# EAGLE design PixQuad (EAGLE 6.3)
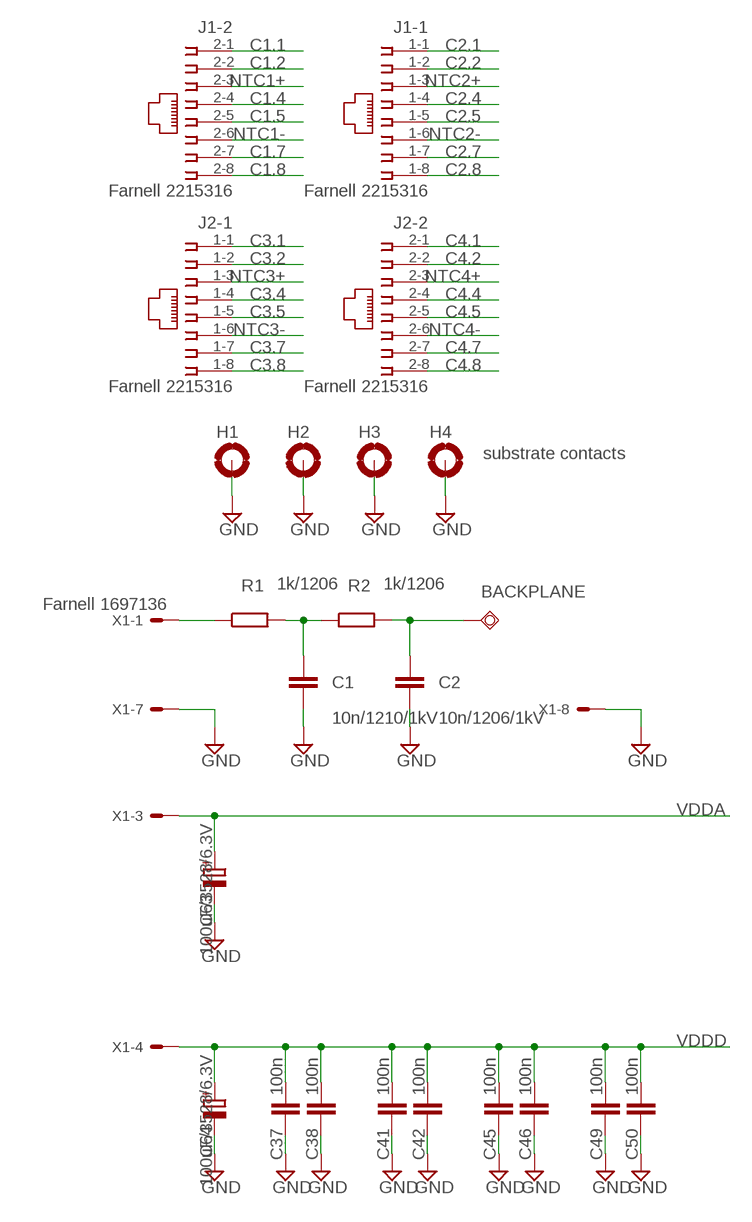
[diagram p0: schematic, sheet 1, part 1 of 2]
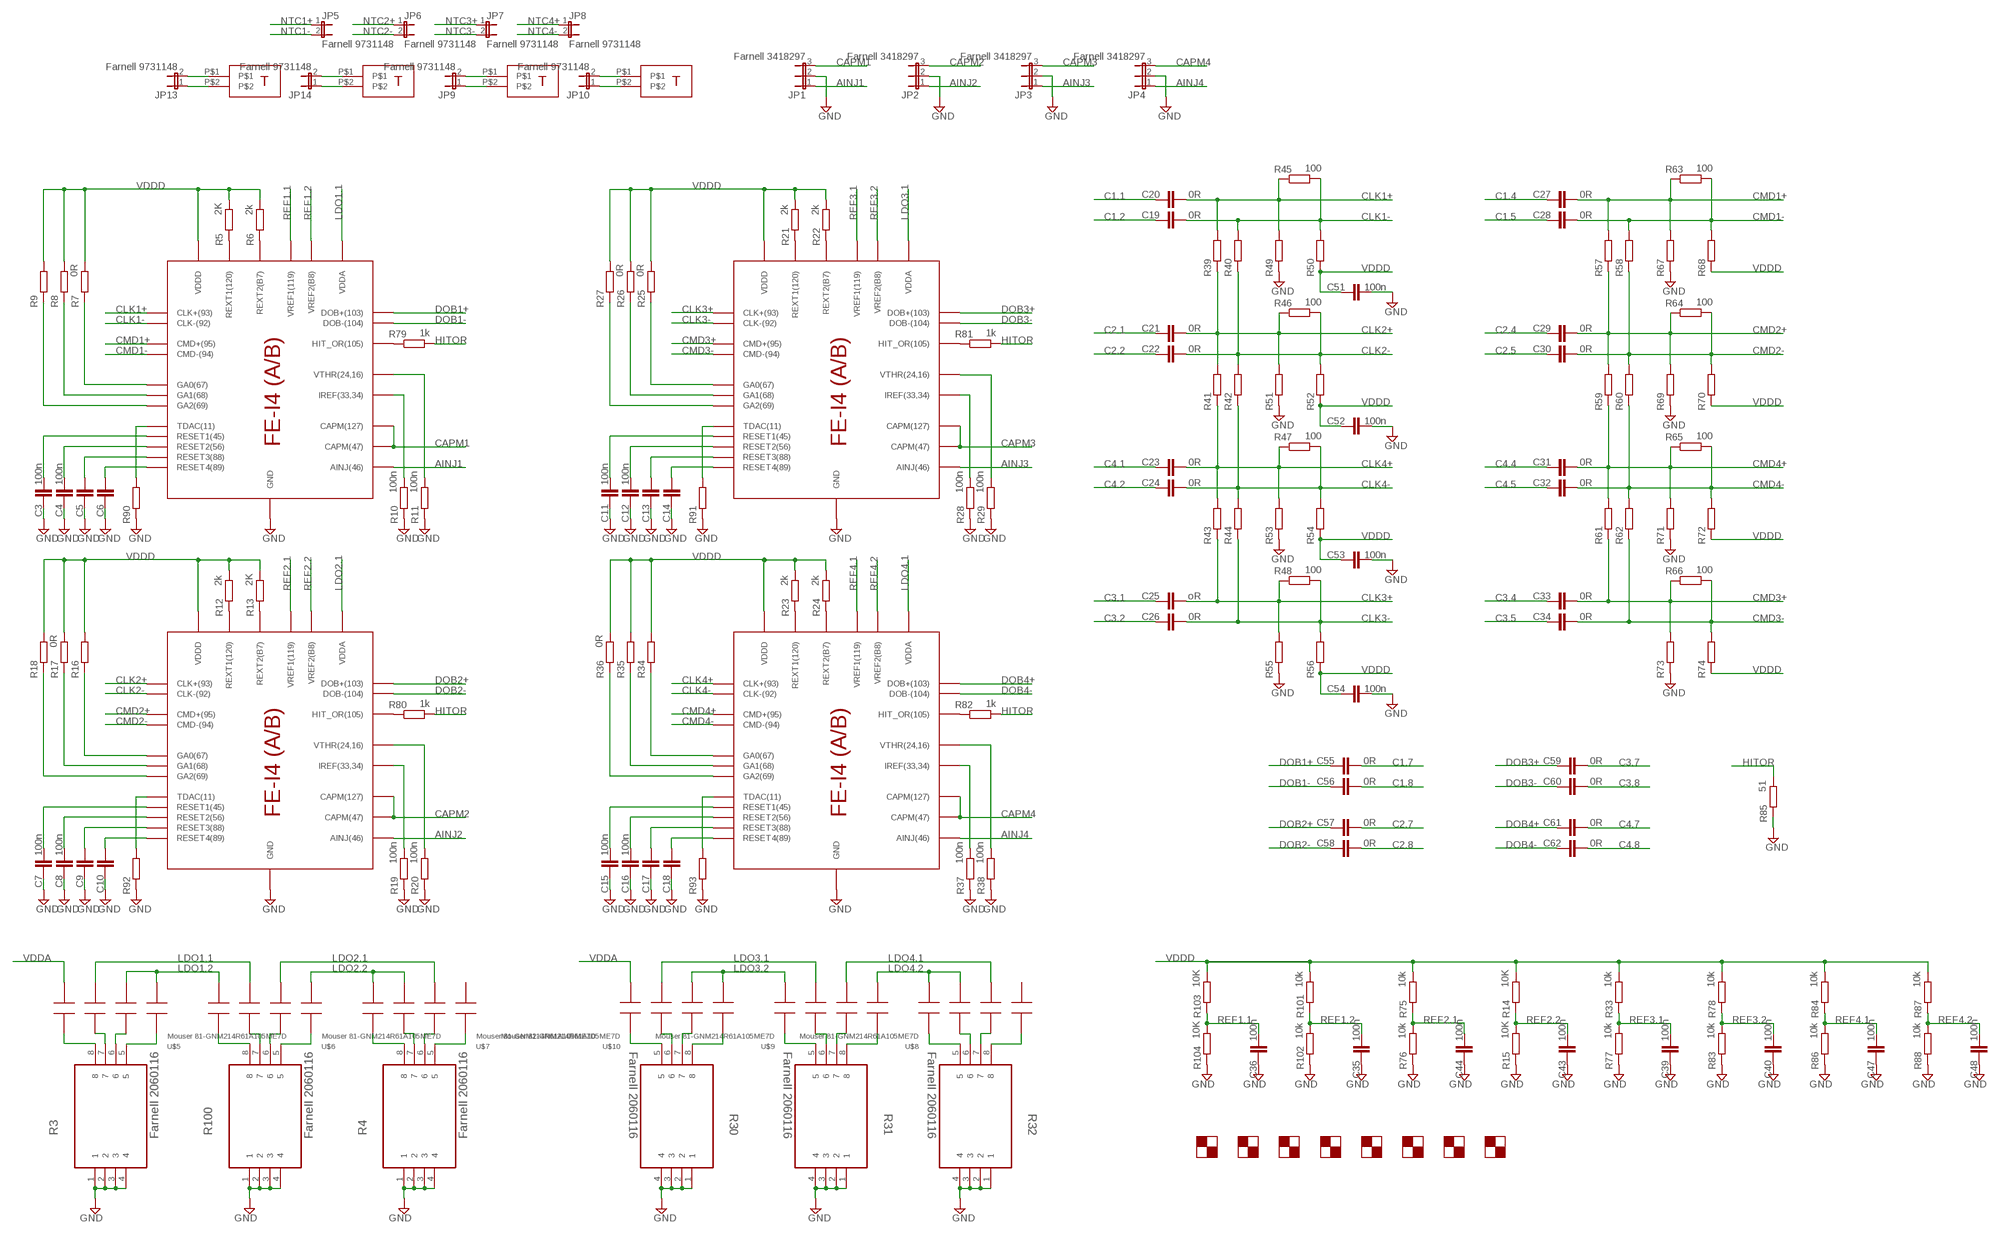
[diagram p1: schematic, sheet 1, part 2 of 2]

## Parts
BACKPLANE  TPSQTP20SQ  [TP20SQ]
C1  10n/1210/1kV  C-EUC1210  [C1210]
C2  10n/1206/1kV  C-EUC1210  [C1210]
C3  100n  C-EUC0402  [C0402]
C4  100n  C-EUC0402  [C0402]
C5  C-EUC0402  [C0402]
C6  C-EUC0402  [C0402]
C7  100n  C-EUC0402  [C0402]
C8  100n  C-EUC0402  [C0402]
C9  C-EUC0402  [C0402]
C10  C-EUC0402  [C0402]
C11  100n  C-EUC0402  [C0402]
C12  100n  C-EUC0402  [C0402]
C13  C-EUC0402  [C0402]
C14  C-EUC0402  [C0402]
C15  100n  C-EUC0402  [C0402]
C16  100n  C-EUC0402  [C0402]
C17  C-EUC0402  [C0402]
C18  C-EUC0402  [C0402]
C19  0R  C-EUC0402  [C0402]
C20  0R  C-EUC0402  [C0402]
C21  0R  C-EUC0402  [C0402]
C22  0R  C-EUC0402  [C0402]
C23  0R  C-EUC0402  [C0402]
C24  0R  C-EUC0402  [C0402]
C25  oR  C-EUC0402  [C0402]
C26  0R  C-EUC0402  [C0402]
C27  0R  C-EUC0402  [C0402]
C28  0R  C-EUC0402  [C0402]
C29  0R  C-EUC0402  [C0402]
C30  0R  C-EUC0402  [C0402]
C31  0R  C-EUC0402  [C0402]
C32  0R  C-EUC0402  [C0402]
C33  0R  C-EUC0402  [C0402]
C34  0R  C-EUC0402  [C0402]
C35  100n  C-EUC0402  [C0402]
C36  100n  C-EUC0402  [C0402]
C37  100n  C-EUC0402  [C0402]
C38  100n  C-EUC0402  [C0402]
C39  100n  C-EUC0402  [C0402]
C40  100n  C-EUC0402  [C0402]
C41  100n  C-EUC0402  [C0402]
C42  100n  C-EUC0402  [C0402]
C43  100n  C-EUC0402  [C0402]
C44  100n  C-EUC0402  [C0402]
C45  100n  C-EUC0402  [C0402]
C46  100n  C-EUC0402  [C0402]
C47  100n  C-EUC0402  [C0402]
C48  100n  C-EUC0402  [C0402]
C49  100n  C-EUC0402  [C0402]
C50  100n  C-EUC0402  [C0402]
C51  100n  C-EUC0402  [C0402]
C52  100n  C-EUC0402  [C0402]
C53  100n  C-EUC0402  [C0402]
C54  100n  C-EUC0402  [C0402]
C55  0R  C-EUC0402  [C0402]
C56  0R  C-EUC0402  [C0402]
C57  0R  C-EUC0402  [C0402]
C58  0R  C-EUC0402  [C0402]
C59  0R  C-EUC0402  [C0402]
C60  0R  C-EUC0402  [C0402]
C61  0R  C-EUC0402  [C0402]
C62  0R  C-EUC0402  [C0402]
C63  100uF/3528/6.3V  CPOL-EUCT3528  [CT3528]
C64  100uF/3528/6.3V  CPOL-EUCT3528  [CT3528]
H1  MOUNT-PAD-ROUND3.2  [3,2-PAD]
H2  MOUNT-PAD-ROUND3.2  [3,2-PAD]
H3  MOUNT-PAD-ROUND3.2  [3,2-PAD]
H4  substrate contacts  MOUNT-PAD-ROUND3.2  [3,2-PAD]
J1  Farnell 2215316  557560-1  [557560-1]
J2  Farnell 2215316  557560-1  [557560-1]
JP1  Farnell 3418297  JP2E  [JP2]
JP2  Farnell 3418297  JP2E  [JP2]
JP3  Farnell 3418297  JP2E  [JP2]
JP4  Farnell 3418297  JP2E  [JP2]
JP5  Farnell 9731148  JP1E  [JP1]
JP6  Farnell 9731148  JP1E  [JP1]
JP7  Farnell 9731148  JP1E  [JP1]
JP8  Farnell 9731148  JP1E  [JP1]
JP9  Farnell 9731148  JP1E  [JUMPER_JP1]
JP10  Farnell 9731148  JP1E  [JUMPER_JP1]
JP13  Farnell 9731148  JP1E  [JUMPER_JP1]
JP14  Farnell 9731148  JP1E  [JUMPER_JP1]
R1  1k/1206  R-EU_R1206  [R1206]
R2  1k/1206  R-EU_R1206  [R1206]
R3  Farnell 2060116  EXB18V100JX  [RESCAF40P140X60X45-8N]
R4  Farnell 2060116  EXB18V100JX  [RESCAF40P140X60X45-8N]
R5  2K  R-EU_R0402  [R0402]
R6  2k  R-EU_R0402  [R0402]
R7  0R  R-EU_R0402  [R0402]
R8  R-EU_R0402  [R0402]
R9  R-EU_R0402  [R0402]
R10  100n  R-EU_R0402  [R0402]
R11  100n  R-EU_R0402  [R0402]
R12  2k  R-EU_R0402  [R0402]
R13  2K  R-EU_R0402  [R0402]
R14  10K  R-EU_R0402  [R0402]
R15  10K  R-EU_R0402  [R0402]
R16  R-EU_R0402  [R0402]
R17  0R  R-EU_R0402  [R0402]
R18  R-EU_R0402  [R0402]
R19  100n  R-EU_R0402  [R0402]
R20  100n  R-EU_R0402  [R0402]
R21  2k  R-EU_R0402  [R0402]
R22  2k  R-EU_R0402  [R0402]
R23  2k  R-EU_R0402  [R0402]
R24  2k  R-EU_R0402  [R0402]
R25  0R  R-EU_R0402  [R0402]
R26  0R  R-EU_R0402  [R0402]
R27  R-EU_R0402  [R0402]
R28  100n  R-EU_R0402  [R0402]
R29  100n  R-EU_R0402  [R0402]
R30  Farnell 2060116  EXB18V100JX  [RESCAF40P140X60X45-8N]
R31  Farnell 2060116  EXB18V100JX  [RESCAF40P140X60X45-8N]
R32  Farnell 2060116  EXB18V100JX  [RESCAF40P140X60X45-8N]
R33  10k  R-EU_R0402  [R0402]
R34  R-EU_R0402  [R0402]
R35  R-EU_R0402  [R0402]
R36  0R  R-EU_R0402  [R0402]
R37  100n  R-EU_R0402  [R0402]
R38  100n  R-EU_R0402  [R0402]
R39  R-EU_R0402  [R0402]
R40  R-EU_R0402  [R0402]
R41  R-EU_R0402  [R0402]
R42  R-EU_R0402  [R0402]
R43  R-EU_R0402  [R0402]
R44  R-EU_R0402  [R0402]
R45  100  R-EU_R0402  [R0402]
R46  100  R-EU_R0402  [R0402]
R47  100  R-EU_R0402  [R0402]
R48  100  R-EU_R0402  [R0402]
R49  R-EU_R0402  [R0402]
R50  R-EU_R0402  [R0402]
R51  R-EU_R0402  [R0402]
R52  R-EU_R0402  [R0402]
R53  R-EU_R0402  [R0402]
R54  R-EU_R0402  [R0402]
R55  R-EU_R0402  [R0402]
R56  R-EU_R0402  [R0402]
R57  R-EU_R0402  [R0402]
R58  R-EU_R0402  [R0402]
R59  R-EU_R0402  [R0402]
R60  R-EU_R0402  [R0402]
R61  R-EU_R0402  [R0402]
R62  R-EU_R0402  [R0402]
R63  100  R-EU_R0402  [R0402]
R64  100  R-EU_R0402  [R0402]
R65  100  R-EU_R0402  [R0402]
R66  100  R-EU_R0402  [R0402]
R67  R-EU_R0402  [R0402]
R68  R-EU_R0402  [R0402]
R69  R-EU_R0402  [R0402]
R70  R-EU_R0402  [R0402]
R71  R-EU_R0402  [R0402]
R72  R-EU_R0402  [R0402]
R73  R-EU_R0402  [R0402]
R74  R-EU_R0402  [R0402]
R75  10k  R-EU_R0402  [R0402]
R76  10k  R-EU_R0402  [R0402]
R77  10k  R-EU_R0402  [R0402]
R78  10k  R-EU_R0402  [R0402]
R79  1k  R-EU_R0402  [R0402]
R80  1k  R-EU_R0402  [R0402]
R81  1k  R-EU_R0402  [R0402]
R82  1k  R-EU_R0402  [R0402]
R83  10k  R-EU_R0402  [R0402]
R84  10k  R-EU_R0402  [R0402]
R85  51  RCL_R-EU_R0603  [RCL_R0603]
R86  10k  R-EU_R0402  [R0402]
R87  10k  R-EU_R0402  [R0402]
R88  10k  R-EU_R0402  [R0402]
R90  R-EU_R0402  [R0402]
R91  R-EU_R0402  [R0402]
R92  R-EU_R0402  [R0402]
R93  R-EU_R0402  [R0402]
R100  Farnell 2060116  EXB18V100JX  [RESCAF40P140X60X45-8N]
R101  10k  R-EU_R0402  [R0402]
R102  10k  R-EU_R0402  [R0402]
R103  10K  R-EU_R0402  [R0402]
R104  10K  R-EU_R0402  [R0402]
U$1  FE_I4ASIC  [FE-I4]
U$2  FE_I4ASIC  [FE-I4]
U$3  FE_I4ASIC  [FE-I4]
U$4  FE_I4ASIC  [FE-I4]
U$5  Mouser 81-GNM214R61A105ME7D  4XC_0508  [4XC_0508]
U$6  Mouser 81-GNM214R61A105ME7D  4XC_0508  [4XC_0508]
U$7  Mouser 81-GNM214R61A105ME7D  4XC_0508  [4XC_0508]
U$8  Mouser 81-GNM214R61A105ME7D  4XC_0508  [4XC_0508]
U$9  Mouser 81-GNM214R61A105ME7D  4XC_0508  [4XC_0508]
U$10  Mouser 81-GNM214R61A105ME7D  4XC_0508  [4XC_0508]
U$11  AMARK  [AMARK]
U$12  AMARK  [AMARK]
U$13  AMARK  [AMARK]
U$14  AMARK  [AMARK]
U$15  AMARK  [AMARK]
U$16  AMARK  [AMARK]
U$17  DORT  [DORT]
U$18  DORT  [DORT]
U$19  AMARK  [AMARK]
U$20  AMARK  [AMARK]
U$21  DORT  [DORT]
U$22  DORT  [DORT]
X1  Farnell 1697136  FE-I4_5566-8  [FE-I4_5566-8]

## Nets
AINJ1: JP1.1 U$1.AINJ(46)
AINJ2: JP2.1 U$2.AINJ(46)
AINJ3: JP3.1 U$3.AINJ(46)
AINJ4: JP4.1 U$4.AINJ(46)
C1.1: C20.2 J1.2-1
C1.2: C19.2 J1.2-2
C1.4: C27.2 J1.2-4
C1.5: C28.2 J1.2-5
C1.7: C55.1 J1.2-7
C1.8: C56.1 J1.2-8
C2.1: C21.2 J1.1-1
C2.2: C22.2 J1.1-2
C2.4: C29.2 J1.1-4
C2.5: C30.2 J1.1-5
C2.7: C57.1 J1.1-7
C2.8: C58.1 J1.1-8
C3.1: C25.2 J2.1-1
C3.2: C26.2 J2.1-2
C3.4: C33.2 J2.1-4
C3.5: C34.2 J2.1-5
C3.7: C59.1 J2.1-7
C3.8: C60.1 J2.1-8
C4.1: C23.2 J2.2-1
C4.2: C24.2 J2.2-2
C4.4: C31.2 J2.2-4
C4.5: C32.2 J2.2-5
C4.7: C61.1 J2.2-7
C4.8: C62.1 J2.2-8
CAPM1: JP1.3 U$1.CAPM(47) U$1.CAPM(125)(CAPM(127))
CAPM2: JP2.3 U$2.CAPM(47) U$2.CAPM(125)(CAPM(127))
CAPM3: JP3.3 U$3.CAPM(47) U$3.CAPM(125)(CAPM(127))
CAPM4: JP4.3 U$4.CAPM(47) U$4.CAPM(125)(CAPM(127))
CLK1+: C20.1 R39.2 R45.1 R49.2 U$1.CLK+(93)
CLK1-: C19.1 R40.2 R45.2 R50.2 U$1.CLK-(92)
CLK2+: C21.1 R39.1 R41.2 R46.1 R51.2 U$2.CLK+(93)
CLK2-: C22.1 R40.1 R42.2 R46.2 R52.2 U$2.CLK-(92)
CLK3+: C25.1 R43.1 R48.1 R55.2 U$3.CLK+(93)
CLK3-: C26.1 R44.1 R48.2 R56.2 U$3.CLK-(92)
CLK4+: C23.1 R41.1 R43.2 R47.1 R53.2 U$4.CLK+(93)
CLK4-: C24.1 R42.1 R44.2 R47.2 R54.2 U$4.CLK-(92)
CMD1+: C27.1 R57.2 R63.1 R67.2 U$1.CMD+(95)
CMD1-: C28.1 R58.2 R63.2 R68.2 U$1.CMD-(94)
CMD2+: C29.1 R57.1 R59.2 R64.1 R69.2 U$2.CMD+(95)
CMD2-: C30.1 R58.1 R60.2 R64.2 R70.2 U$2.CMD-(94)
CMD3+: C33.1 R61.1 R66.1 R73.2 U$3.CMD+(95)
CMD3-: C34.1 R62.1 R66.2 R74.2 U$3.CMD-(94)
CMD4+: C31.1 R59.1 R61.2 R65.1 R71.2 U$4.CMD+(95)
CMD4-: C32.1 R60.1 R62.2 R65.2 R72.2 U$4.CMD-(94)
DOB1+: C55.2 U$1.DOB+(103)
DOB1-: C56.2 U$1.DOB-(104)
DOB2+: C57.2 U$2.DOB+(103)
DOB2-: C58.2 U$2.DOB-(104)
DOB3+: C59.2 U$3.DOB+(103)
DOB3-: C60.2 U$3.DOB-(104)
DOB4+: C61.2 U$4.DOB+(103)
DOB4-: C62.2 U$4.DOB-(104)
GND: C1.2 C2.2 C3.2 C4.2 C5.2 C6.2 C7.2 C8.2 C9.2 C10.2 C11.2 C12.2 C13.2 C14.2 C15.2 C16.2 C17.2 C18.2 C35.2 C36.2 C37.2 C38.2 C39.2 C40.2 C41.2 C42.2 C43.2 C44.2 C45.2 C46.2 C47.2 C48.2 C49.2 C50.2 C51.1 C52.1 C53.1 C54.1 C63.- C64.- H1.B3,2(MOUNT) H2.B3,2(MOUNT) H3.B3,2(MOUNT) H4.B3,2(MOUNT) JP1.2 JP2.2 JP3.2 JP4.2 R3.1 R3.2 R3.3 R3.4 R4.1 R4.2 R4.3 R4.4 R10.1 R11.1 R15.1 R19.1 R20.1 R28.1 R29.1 R30.1 R30.2 R30.3 R30.4 R31.1 R31.2 R31.3 R31.4 R32.1 R32.2 R32.3 R32.4 R37.1 R38.1 R49.1 R51.1 R53.1 R55.1 R67.1 R69.1 R71.1 R73.1 R76.1 R77.1 R83.1 R85.1 R86.1 R88.1 R90.1 R91.1 R92.1 R93.1 R100.1 R100.2 R100.3 R100.4 R102.1 R104.1 U$1.GND U$2.GND U$3.GND U$4.GND X1.7 X1.8
HITOR: R79.2 R80.2 R81.2 R82.2 R85.2
LDO1.1: U$1.VDDA U$5.P$4 U$6.P$4
LDO1.2: U$5.P$6 U$5.P$8 U$6.P$2
LDO2.1: U$2.VDDA U$6.P$6 U$7.P$6
LDO2.2: U$6.P$8 U$7.P$2 U$7.P$4
LDO3.1: U$3.VDDA U$9.P$6 U$10.P$6
LDO3.2: U$9.P$8 U$10.P$2 U$10.P$4
LDO4.1: U$4.VDDA U$8.P$4 U$9.P$4
LDO4.2: U$8.P$6 U$8.P$8 U$9.P$2
N$1: BACKPLANE.TP C2.1 R2.2
N$2: C1.1 R1.2 R2.1
N$3: JP13.2 U$17.P$1
N$4: C3.1 U$1.RESET1(45)
N$5: C4.1 U$1.RESET2(56)
N$6: C5.1 U$1.RESET3(88)
N$7: C6.1 U$1.RESET4(89)
N$8: R7.1 U$1.GA0(67)
N$9: R8.1 U$1.GA1(68)
N$10: R9.1 U$1.GA2(69)
N$11: R10.2 U$1.IREF(33,34)
N$12: R11.2 U$1.VTHR(24,16)
N$13: R79.1 U$1.HITOR(105)(HIT_OR(105))
N$14: R16.1 U$2.GA0(67)
N$15: R17.1 U$2.GA1(68)
N$16: R18.1 U$2.GA2(69)
N$17: C7.1 U$2.RESET1(45)
N$18: C8.1 U$2.RESET2(56)
N$19: C9.1 U$2.RESET3(88)
N$20: C10.1 U$2.RESET4(89)
N$21: R80.1 U$2.HITOR(105)(HIT_OR(105))
N$22: R81.1 U$3.HITOR(105)(HIT_OR(105))
N$23: R82.1 U$4.HITOR(105)(HIT_OR(105))
N$24: R90.2 U$1.TDAC(11)
N$25: R19.2 U$2.IREF(33,34)
N$26: R20.2 U$2.VTHR(24,16)
N$27: R91.2 U$3.TDAC(11)
N$28: R92.2 U$2.TDAC(11)
N$29: R93.2 U$4.TDAC(11)
N$30: JP13.1 U$17.P$2
N$31: JP14.1 U$18.P$2
N$32: JP14.2 U$18.P$1
N$33: R3.8 U$5.P$1
N$34: R1.1 X1.1
N$35: R12.1 U$2.REXT1(120)
N$38: R3.5 U$5.P$7
N$39: R3.7 U$5.P$3
N$40: R3.6 U$5.P$5
N$41: R100.8 U$6.P$1
N$42: R100.7 U$6.P$3
N$43: R100.6 U$6.P$5
N$44: R100.5 U$6.P$7
N$45: R4.8 U$7.P$1
N$46: JP9.1 U$21.P$2
N$47: JP9.2 U$21.P$1
N$48: JP10.1 U$22.P$2
N$49: JP10.2 U$22.P$1
N$50: R27.1 U$3.GA2(69)
N$51: R5.1 U$1.REXT1(120)
N$52: R6.1 U$1.REXT2(B7)
N$53: R4.7 U$7.P$3
N$54: R4.6 U$7.P$5
N$55: R4.5 U$7.P$7
N$56: R28.2 U$3.IREF(33,34)
N$57: R26.1 U$3.GA1(68)
N$58: R25.1 U$3.GA0(67)
N$59: C11.1 U$3.RESET1(45)
N$60: C12.1 U$3.RESET2(56)
N$61: C13.1 U$3.RESET3(88)
N$62: C14.1 U$3.RESET4(89)
N$63: R13.1 U$2.REXT2(B7)
N$64: R29.2 U$3.VTHR(24,16)
N$65: R21.1 U$3.REXT1(120)
N$66: R22.1 U$3.REXT2(B7)
N$67: R23.1 U$4.REXT1(120)
N$68: R24.1 U$4.REXT2(B7)
N$69: R30.5 U$10.P$7
N$70: R30.8 U$10.P$1
N$71: R30.6 U$10.P$5
N$72: R30.7 U$10.P$3
N$73: R34.1 U$4.GA0(67)
N$74: R35.1 U$4.GA1(68)
N$75: R36.1 U$4.GA2(69)
N$76: C15.1 U$4.RESET1(45)
N$77: C16.1 U$4.RESET2(56)
N$78: C17.1 U$4.RESET3(88)
N$79: C18.1 U$4.RESET4(89)
N$80: R37.2 U$4.IREF(33,34)
N$81: R38.2 U$4.VTHR(24,16)
N$82: R31.6 U$9.P$5
N$83: R31.5 U$9.P$7
N$84: R31.8 U$9.P$1
N$85: R31.7 U$9.P$3
N$86: R32.5 U$8.P$7
N$87: R32.6 U$8.P$5
N$88: R32.7 U$8.P$3
N$89: R32.8 U$8.P$1
NTC1+: J1.2-3 JP5.1
NTC1-: J1.2-6 JP5.2
NTC2+: J1.1-3 JP6.1
NTC2-: J1.1-6 JP6.2
NTC3+: J2.1-3 JP7.1
NTC3-: J2.1-6 JP7.2
NTC4+: J2.2-3 JP8.1
NTC4-: J2.2-6 JP8.2
REF1.1: C36.1 R103.1 R104.2 U$1.VREF1(119)
REF1.2: C35.1 R101.1 R102.2 U$1.VREF2(B8)
REF2.1: C44.1 R75.1 R76.2 U$2.VREF1(119)
REF2.2: C43.1 R14.1 R15.2 U$2.VREF2(B8)
REF3.1: C39.1 R33.1 R77.2 U$3.VREF1(119)
REF3.2: C40.1 R78.1 R83.2 U$3.VREF2(B8)
REF4.1: C47.1 R84.1 R86.2 U$4.VREF1(119)
REF4.2: C48.1 R87.1 R88.2 U$4.VREF2(B8)
VDDA: C63.+ U$5.P$2 U$10.P$8 X1.3
VDDD: C37.1 C38.1 C41.1 C42.1 C45.1 C46.1 C49.1 C50.1 C51.2 C52.2 C53.2 C54.2 C64.+ R5.2 R6.2 R7.2 R8.2 R9.2 R12.2 R13.2 R14.2 R16.2 R17.2 R18.2 R21.2 R22.2 R23.2 R24.2 R25.2 R26.2 R27.2 R33.2 R34.2 R35.2 R36.2 R50.1 R52.1 R54.1 R56.1 R68.1 R70.1 R72.1 R74.1 R75.2 R78.2 R84.2 R87.2 R101.2 R103.2 U$1.VDDD U$2.VDDD U$3.VDDD U$4.VDDD X1.4
Unconnected: U$7.P$8 U$8.P$2

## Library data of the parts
BACKPLANE = testpad:TPSQ: Test pad
C1-C62 = rcl:C-EU: CAPACITOR, European symbol
C63 C64 = rcl:CPOL-EU: POLARIZED CAPACITOR, European symbol
H1-H4 = holes:MOUNT-PAD-ROUND: MOUNTING PAD, round
J1 J2 = con-amp:557560-1: AMP connector
JP1-JP4 = jumper:JP2E: JUMPER
JP5-JP8 = jumper:JP1E: JUMPER
JP9 JP10 JP13 JP14 = FE-I4:JP1E: JUMPER
R1 R2 R5-R29 R33-R84 R86-R88 R90-R93 R101-R104 = rcl:R-EU_: RESISTOR, European symbol
R3 R4 R30-R32 R100 = Panasonic-EXB-ERJ:EXB18V: Chip Resistor Array; MPN: EXB18V100JX; OC_FARNELL: 2060116; OC_NEWARK: 65T9021; PACKAGE: 0201; POWERRATING: wattage 0.031 W/element (0.1 W/package); SUPPLIER: PANASONIC; TOLERANCE: ±5 %; VALUE: 10R
R85 = FE-I4:RCL_R-EU_: RESISTOR, European symbol
U$1-U$4 = FE-I4:FE_I4
U$5-U$10 = FE-I4:4XC_0508; C: 100n
U$11-U$16 U$19 U$20 = FE-I4:AMARK
U$17 U$18 U$21 U$22 = FE-I4:DORT
X1 = FE-I4:FE-I4_5566-8: Mini FIT connector 8 pol Source: http://www.molex.com; OC_FARNELL: unknown; OC_NEWARK: unknown

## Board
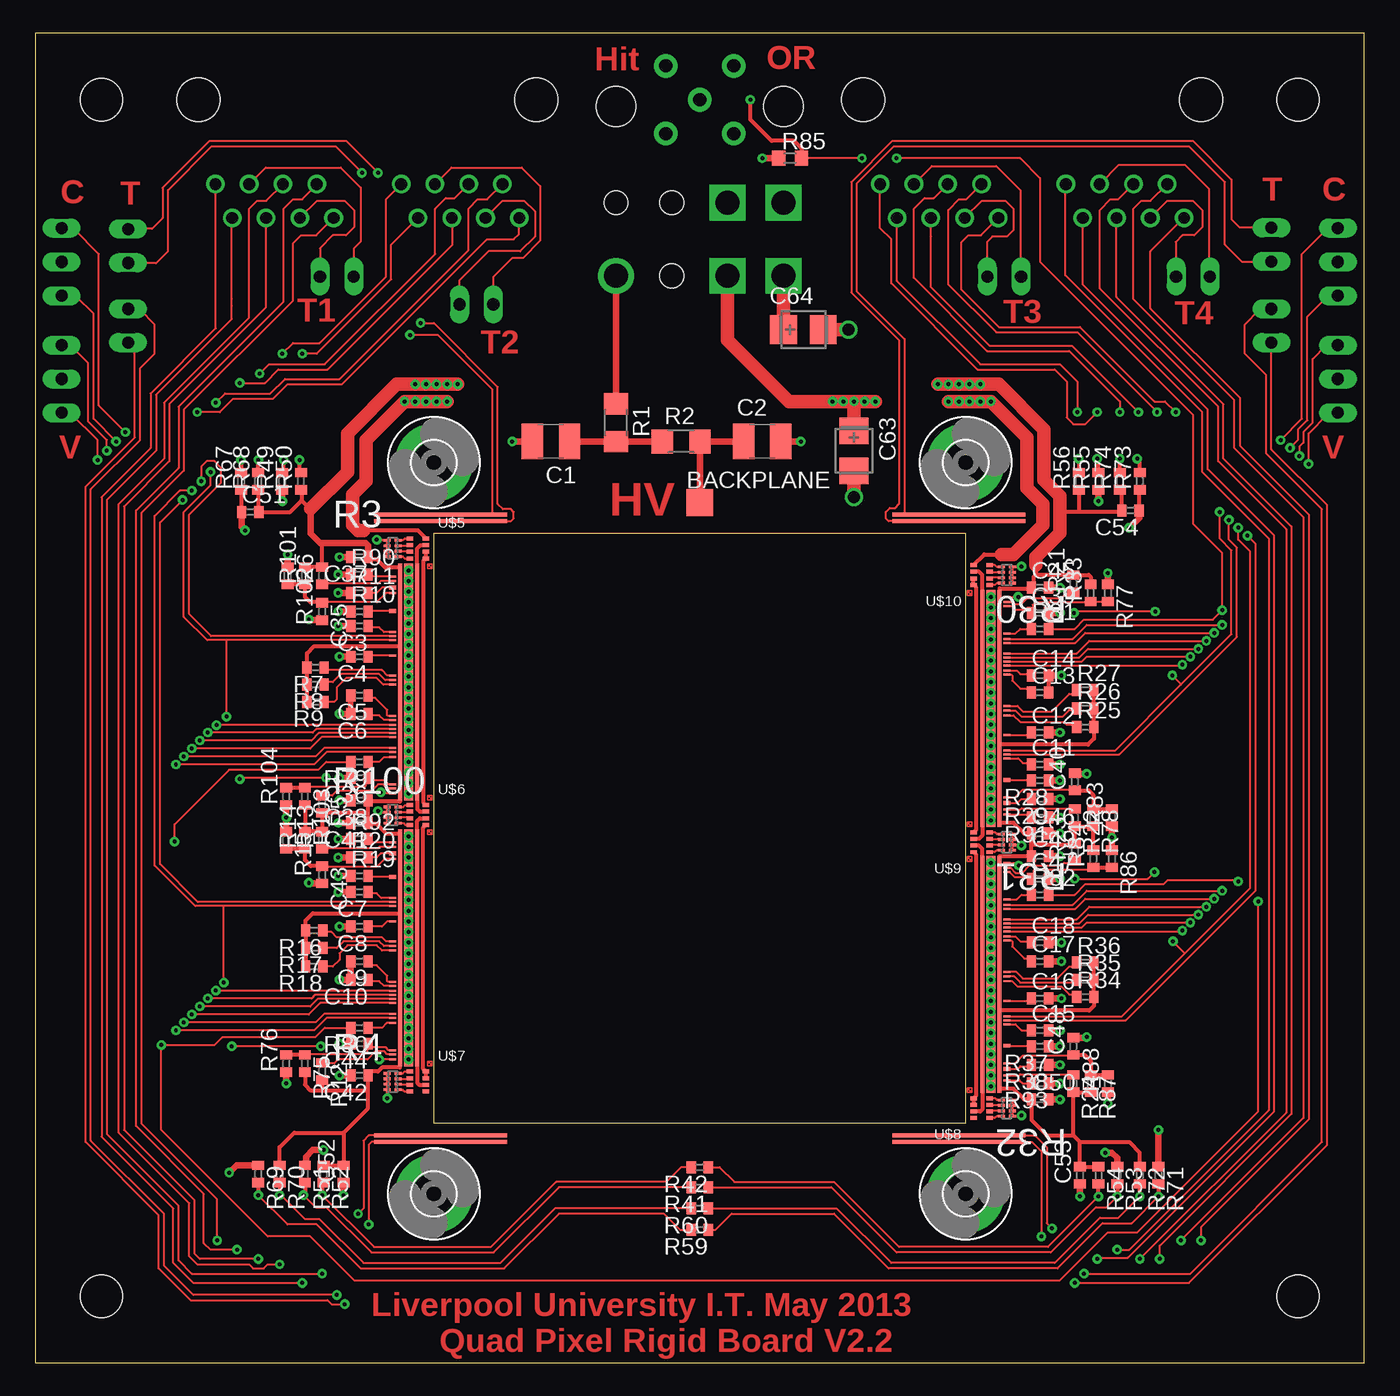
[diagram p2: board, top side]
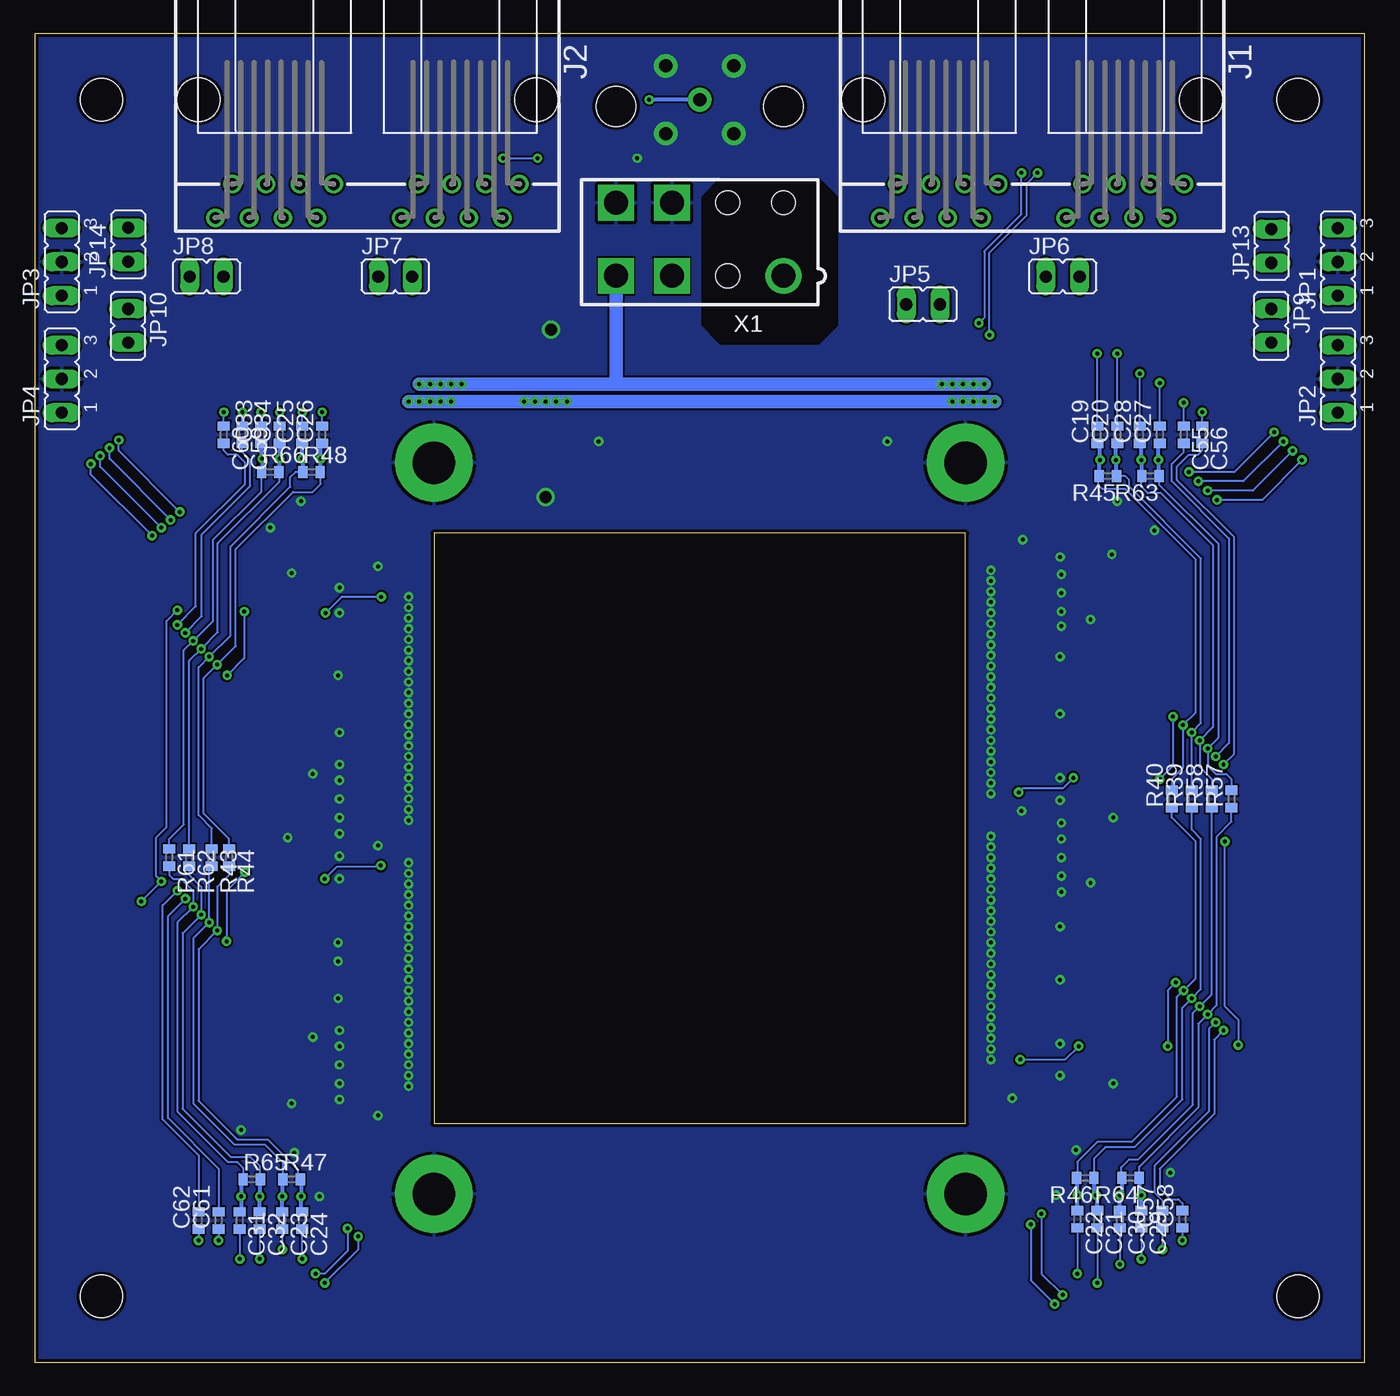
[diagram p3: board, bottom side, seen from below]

Size 100 x 100 mm. Coordinates in mm from the lower left corner, seen from the top.
Outline: 0,0 100,0 100,100 0,100 0,0
Copper layers (1+2*15+16): Top 0.035mm / dielectric 1.5mm / Route2 0.035mm / dielectric 0.15mm / Route15 0.035mm / dielectric 0.2mm / Bottom 0.035mm
Design rules "default *": minimum track width 10mil, minimum drill 24mil, track to track 6mil, track to pad 6mil, pad to pad 6mil, via to via 6mil, smd to smd 6mil, copper to edge 10mil, drill to drill 8mil, minimum pad ring 10mil, minimum via ring 8mil, stop-mask expansion 4mil, vias tented up to drill 0mil, thermal gap 10mil
Holes 3.2 mm at 5,5 5,95 95,95 95,5

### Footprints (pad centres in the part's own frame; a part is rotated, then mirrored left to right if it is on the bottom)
TP20SQ = smd 2 x 2: TP 0,0
C1210 = smd 1.6 x 2.7: 1 -1.4,0; 2 1.4,0
C0402 = smd 0.7 x 0.9: 1 -0.65,0; 2 0.65,0
CT3528 = smd 2 x 2.2: + -1.5,0; - 1.5,0
3,2-PAD = drill 3.2 pad 5.842: B3,2 0,0
557560-1 = drill 0.889: 1-1 -11.43,6.35; 1-2 -10.16,8.89; 1-3 -8.89,6.35; 1-4 -7.62,8.89; 1-5 -6.35,6.35; 1-6 -5.08,8.89; 1-7 -3.81,6.35; 1-8 -2.54,8.89; 2-1 2.54,6.35; 2-2 3.81,8.89; 2-3 5.08,6.35; 2-4 6.35,8.89; 2-5 7.62,6.35; 2-6 8.89,8.89; 2-7 10.16,6.35; 2-8 11.43,8.89 | hole 3.251: -12.7,0; 12.7,0
JP2 = drill 0.914 long: 1 -2.54,0; 2 0,0; 3 2.54,0
JP1 = drill 0.914 long: 1 0,-1.27; 2 0,1.27
JUMPER_JP1 = drill 0.914 long: 1 0,-1.27; 2 0,1.27
R1206 = smd 1.6 x 1.803: 1 -1.422,0; 2 1.422,0
RESCAF40P140X60X45-8N = smd 0.508 x 0.203: 1 -0.406,0.61; 2 -0.406,0.203; 3 -0.406,-0.203; 4 -0.406,-0.61; 5 0.406,-0.61; 6 0.406,-0.203; 7 0.406,0.203; 8 0.406,0.61
R0402 = smd 0.7 x 0.9: 1 -0.65,0; 2 0.65,0
RCL_R0603 = smd 1 x 1.1: 1 -0.85,0; 2 0.85,0
FE-I4 = smd 0.15 x 0.5: AINJ(46) -4.45,-2; CAPM(47) -4.15,-2; CAPM(125) 7.4,-2; CLK+(93) 2.55,-2; CLK-(92) 2.25,-2; CMD+(95) 3.15,-2; CMD-(94) 2.85,-2; DOB+(103) 3.95,-2; DOB-(104) 4.25,-2; GA0(67) -1.5,-2; GA1(68) -1.15,-2; GA2(69) -0.8,-2; HITOR(105) 4.65,-2; RESET1(45) -4.75,-2; RESET2(56) -3,-2; RESET3(88) 1.55,-2; RESET4(89) 1.85,-2; REXT1(120) 7,-2; REXT2(B7) -8.6,-2; TDAC(11) -8.95,-2; VREF1(119) 6.7,-2; VREF2(B8) -7.7,-2 | smd 17.8 x 0.7: GND -1,-0.8 | smd 0.3 x 0.5: IREF(33,34) -6.35,-2; VTHR(24,16) -8.1,-2 | smd 17.8 x 0.3: VDDA -1,-0.15; VDDD -1,-1.45
4XC_0508 = smd 0.5 x 0.3: P$1 0,0; P$2 1.2,0; P$3 0,-0.5; P$4 1.2,-0.5; P$5 0,-1; P$6 1.2,-1; P$7 0,-1.5; P$8 1.2,-1.5
DORT = smd 10 x 0.3: P$1 5,0; P$2 5,0.5
FE-I4_5566-8 = drill 1.8: 1 6.3,-2.75 | drill 1.8 square: 3 -2.1,-2.75; 4 -6.3,-2.75; 7 -2.1,2.75; 8 -6.3,2.75 | hole 1.8: 2.1,-2.75; 2.1,2.75; 6.3,2.75 | hole 3: -6.3,10; 6.3,10

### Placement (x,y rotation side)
BACKPLANE  50,64.7 0 top
C1  38.8,69.3 180 top
C2  54.7,69.3 0 top
C3  24.4,55.4 180 top
C4  24.4,53.1 180 top
C5  24.4,50.2 180 top
C6  24.4,48.8 180 top
C7  24.4,35.4 180 top
C8  24.4,32.8 180 top
C9  24.4,30.2 180 top
C10  24.4,28.8 180 top
C11  75.6,45 0 top
C12  75.6,47.4 0 top
C13  75.6,50.4 0 top
C14  75.6,51.7 0 top
C15  75.6,25 0 top
C16  75.6,27.4 0 top
C17  75.6,30.2 0 top
C18  75.6,31.6 0 top
C19  20.1,69.8 90 bottom
C20  18.6,69.8 90 bottom
C21  20.1,10.8 270 bottom
C22  21.6,10.8 270 bottom
C23  81.4,10.7 270 bottom
C24  79.9,10.7 270 bottom
C25  79.9,69.8 90 bottom
C26  78.4,69.8 90 bottom
C27  15.4,69.8 90 bottom
C28  16.9,69.8 90 bottom
C29  16.8,10.8 270 bottom
C30  18.4,10.8 270 bottom
C31  84.6,10.7 270 bottom
C32  83.1,10.7 270 bottom
C33  83,69.8 90 bottom
C34  81.6,69.8 90 bottom
C35  21.6,56.5 270 top
C36  24.4,44 180 top
C37  24.4,60.6 180 top
C38  24.4,42.3 180 top
C39  75.6,56.4 0 top
C40  78.2,43.7 90 top
C41  24.4,40.6 180 top
C42  24.4,21.6 180 top
C43  21.6,36.7 270 top
C44  24.4,24 180 top
C45  75.6,58.3 0 top
C46  75.6,39.8 0 top
C47  75.6,36.4 0 top
C48  78.1,23.8 90 top
C49  75.6,38.1 0 top
C50  75.6,19.8 0 top
C51  16.2,64 0 top
C52  23.2,14.2 90 top
C53  78.6,14.1 90 top
C54  82.4,64.1 180 top
C55  13.6,69.8 270 bottom
C56  12.2,69.8 270 bottom
C57  15.2,10.8 90 bottom
C58  13.7,10.8 90 bottom
C59  84.4,69.8 270 bottom
C60  85.8,69.8 270 bottom
C61  86.2,10.7 90 bottom
C62  87.7,10.7 90 bottom
C63  61.6,68.6 270 top
C64  57.8,77.7 0 top
H1  30,67.7 0 top
H2  30,12.7 0 top
H3  70,67.7 0 top
H4  70,12.7 0 top
J1  25,95 180 bottom
J2  75,95 180 bottom
JP1  2,82.8 90 bottom
JP2  2,74 90 bottom
JP3  98,82.8 90 bottom
JP4  98,74 90 bottom
JP5  33.2,79.6 270 bottom
JP6  22.7,81.7 270 bottom
JP7  72.9,81.7 270 bottom
JP8  87.1,81.7 270 bottom
JP9  7,78 180 bottom
JP10  93,78 180 bottom
JP13  7,84 0 bottom
JP14  93,84.1 0 bottom
R1  43.7,70.7 270 top
R2  48.6,69.3 0 top
R3  26.9,61.25 0 top
R4  26.9,21.15 0 top
R5  21.6,42 270 top
R6  21.6,59.2 90 top
R7  21.1,52.3 180 top
R8  21.1,51 180 top
R9  21.1,49.7 180 top
R10  24.4,56.5 0 top
R11  24.4,57.9 0 top
R12  21.6,21.9 270 top
R13  21.6,39.3 90 top
R14  20.3,39.3 90 top
R15  18.9,39.3 270 top
R16  21,32.5 180 top
R17  21,31.2 180 top
R18  21,29.8 180 top
R19  24.4,36.6 0 top
R20  24.4,38 0 top
R21  78.1,58.6 90 top
R22  78.2,41 270 top
R23  78.2,38.4 90 top
R24  78.1,21 270 top
R25  79,47.8 0 top
R26  79,49.2 0 top
R27  79,50.6 0 top
R28  75.6,43.8 180 top
R29  75.6,42.4 180 top
R30  73.1,59.25 180 top
R31  73.1,39.15 180 top
R32  73.1,19.15 180 top
R33  79.4,57.9 90 top
R34  79,27.5 0 top
R35  79,28.8 0 top
R36  79,30.1 0 top
R37  75.6,23.8 180 top
R38  75.6,22.4 180 top
R39  13,42.4 90 bottom
R40  14.5,42.4 90 bottom
R41  50,13.2 180 top
R42  50,14.7 180 top
R43  86.7,38 270 bottom
R44  85.4,38 270 bottom
R45  19.3,66.7 180 bottom
R46  21,13.9 180 bottom
R47  80.7,13.8 0 bottom
R48  79.2,67 0 bottom
R49  18.6,66.3 90 top
R50  20,66.3 90 top
R51  20.3,14.2 270 top
R52  21.7,14.2 270 top
R53  81.4,14.1 270 top
R54  80,14.1 270 top
R55  80,66.3 90 top
R56  78.5,66.3 90 top
R57  10,42.4 90 bottom
R58  11.5,42.4 90 bottom
R59  50,10 180 top
R60  50,11.6 180 top
R61  89.9,38 270 bottom
R62  88.4,38 270 bottom
R63  16.1,66.7 180 bottom
R64  17.6,13.9 180 bottom
R65  83.7,13.8 0 bottom
R66  82.3,67 0 bottom
R67  15.5,66.3 90 top
R68  16.8,66.3 90 top
R69  16.8,14.2 270 top
R70  18.4,14.2 270 top
R71  84.5,14.1 270 top
R72  83.1,14.1 270 top
R73  83.1,66.3 90 top
R74  81.6,66.3 90 top
R75  20.3,22.5 270 top
R76  18.9,22.5 90 top
R77  80.7,57.9 270 top
R78  79.6,41 270 top
R79  24.4,45.2 180 top
R80  24.4,25.2 180 top
R81  75.6,55.2 0 top
R82  75.6,35.2 0 top
R83  81,41 90 top
R84  79.6,37.9 90 top
R85  56.8,90.6 0 top
R86  81,37.9 270 top
R87  79.4,21 270 top
R88  80.7,21 90 top
R90  24.4,59.3 0 top
R91  75.6,41 180 top
R92  24.4,39.4 0 top
R93  75.6,21 180 top
R100  26.9,41.2 0 top
R101  20.3,59.2 90 top
R102  19,59.2 270 top
R103  20.3,42.6 270 top
R104  18.9,42.6 90 top
U$1  28.9,50.2 270 top
U$2  28.9,30.2 270 top
U$3  71.1,50.2 90 top
U$4  71.1,30.2 90 top
U$5  28.2,62 0 top
U$6  28.2,41.95 0 top
U$7  28.2,21.9 0 top
U$8  71.8,18.4 180 top
U$9  71.8,38.4 180 top
U$10  71.8,58.5 180 top
U$11  29.7,39.9 0 top
U$12  29.7,42.5 0 top
U$13  29.7,59.9 0 top
U$14  70.3,20.5 0 top
U$15  70.3,37.9 0 top
U$16  70.3,40.5 0 top
U$17  25.5,63.3 0 top
U$18  64.5,63.3 0 top
U$19  70.3,57.9 0 top
U$20  29.7,22.5 0 top
U$21  25.5,16.6 0 top
U$22  64.5,16.6 0 top
X1  50,84.5 0 bottom

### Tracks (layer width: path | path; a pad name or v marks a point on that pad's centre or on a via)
AINJ1  (via drill 0.3)
  Top 0.15: U$1.AINJ(46) 13.25,54.65 11.6,56.3 11.6,63.8 14,66.2 14,67.3 13.5,67.8 12.9,67.8 12.5,67.4 v12.5,66.3 | v6.1,69.3 4.4,71 4.4,78.9 3.1,80.2 2.06,80.2 JP1.1
  Bottom 0.15: v6.1,69.3 9.1,66.3 v12.5,66.3
AINJ2  (via drill 0.3)
  Top 0.15: U$2.AINJ(46) 12.25,34.65 9.4,37.5 9.4,63.2 v11.1,64.9 | v4.7,67.9 4.7,69.4 2.7,71.4 2.06,71.4 JP2.1
  Bottom 0.15: v4.7,67.9 7.7,64.9 v11.1,64.9
AINJ3  (via drill 0.3)
  Top 0.15: v89.8,63.4 89.8,61.9 90.4,61.3 90.4,54.6 81.55,45.75 U$3.AINJ(46) | v94.4,68.8 95,69.4 95,70.2 95.7,70.9 95.7,78.7 97.2,80.2 97.94,80.2 JP3.1
  Bottom 0.15: v89.8,63.4 94.4,68 v94.4,68.8
AINJ4  (via drill 0.3)
  Top 0.15: U$4.AINJ(46) 82.05,25.75 91.8,35.5 91.8,61.6 v91.2,62.2 | v95.8,67.6 95.8,69.9 97.2,71.3 97.84,71.3 JP4.1
  Bottom 0.15: v91.2,62.2 95.8,66.8 v95.8,67.6
C1.1  (via drill 0.3)
  Top 0.15: v18.6,75.9 19.4,76.7 21.4,76.7 26.4,81.7 26.4,87.51 J1.2-1 27.5,88.61
  Bottom 0.15: C20.2 v18.6,75.9
C1.2  (via drill 0.3)
  Top 0.15: J1.2-2 26.8,84.1 26.8,81.5 21.2,75.9 v20.1,75.9
  Bottom 0.15: C19.2 v20.1,75.9
C1.4  (via drill 0.3)
  Top 0.15: v15.4,73.7 17.3,73.7 18.3,74.7 22,74.7 31.4,84.1 31.4,86.06 J1.2-4
  Bottom 0.15: C27.2 v15.4,73.7
C1.5  (via drill 0.3)
  Top 0.15: v16.9,74.4 17.6,75.1 21.8,75.1 30.1,83.4 30.1,86.8 30.9,87.6 31.57,87.6 J1.2-5
  Bottom 0.15: C28.2 v16.9,74.4
C1.7  (via drill 0.3)
  Top 0.15: v13.6,72.2 14.3,72.9 17.7,72.9 18.8,74 22.9,74 32.6,83.7 32.6,86.8 33.3,87.5 34.01,87.5 J1.2-7
  Bottom 0.15: C55.1 v13.6,72.2
C1.8  (via drill 0.3)
  Top 0.15: v12.2,71.5 13.9,71.5 14.9,72.5 17.9,72.5 19,73.6 23.1,73.6 34,84.5 36,84.5 36.4,84.9 36.4,86.08 J1.2-8
  Bottom 0.15: C56.1 v12.2,71.5
C2.1  (via drill 0.3)
  Top 0.15: J1.1-1 13.6,88.62 13.6,77.8 8.7,72.9 8.7,68.8 5,65.1 5,17 10.4,11.6 10.4,7.5 11.9,6 v20.1,6
  Bottom 0.15: C21.2 v20.1,6
C2.2  (via drill 0.3)
  Top 0.15: J1.1-2 14.8,86.07 14.8,80 14.8,79.5 14.8,78.5 9.1,72.8 9.1,68.6 5.4,64.9 5.4,17.2 10.8,11.8 10.8,7.7 11.8,6.7 v21.6,6.7
  Bottom 0.15: C22.2 v21.6,6.7
C2.4  (via drill 0.3)
  Top 0.15: v16.8,7.8 12.4,7.8 12,8.2 12,12.2 6.7,17.5 6.7,64.4 10.1,67.8 10.1,72.1 17.38,79.38 17.38,80.38 17.38,80.9 J1.1-4
  Bottom 0.15: C29.2 v16.8,7.8
C2.5  (via drill 0.3)
  Top 0.15: v18.4,7.4 17.5,7.4 17.2,7.1 16.4,7.1 16.1,7.4 12.2,7.4 11.6,8 11.6,12 6.3,17.3 6.3,64.6 9.7,68 9.7,72.2 16.1,78.6 16.1,86.8 16.7,87.4 17.4,87.4 J1.1-5
  Bottom 0.15: C30.2 v18.4,7.4
C2.7  (via drill 0.3)
  Top 0.15: v15.2,8.5 13.2,8.5 12.7,9 12.7,12.7 7.6,17.8 7.6,64.1 10.8,67.3 10.8,71.9 18.7,79.8 18.7,86.8 19.4,87.5 20.1,87.5 21.19,88.59 J1.1-7
  Bottom 0.15: C57.1 v15.2,8.5
C2.8  (via drill 0.3)
  Top 0.15: J1.1-8 21.15,84.8 20,84.8 19.4,84.2 19.4,81 19.4,80.7 19.4,79.9 11.2,71.7 11.2,67.1 8,63.9 8,18 13.7,12.3 v13.7,9.2
  Bottom 0.15: C58.1 v13.7,9.2
C3.1  (via drill 0.3)
  Top 0.15: v79.9,71.5 79,70.6 78.1,70.6 77.6,71.1 77.6,73.8 76.7,74.7 70.9,74.7 64.4,81.2 64.4,84.5 63.57,85.33 J2.1-1
  Bottom 0.15: C25.2 v79.9,71.5
C3.2  (via drill 0.3)
  Top 0.15: J2.1-2 64.84,81.36 71.1,75.1 77.1,75.1 78.4,73.8 v78.4,71.5
  Bottom 0.15: C26.2 v78.4,71.5
C3.4  (via drill 0.3)
  Top 0.15: J2.1-4 67.38,84.72 67.4,84.7 67.4,80.9 71.8,76.5 78,76.5 v83,71.5
  Bottom 0.15: C33.2 v83,71.5
C3.5  (via drill 0.3)
  Top 0.15: v81.6,71.5 81.6,72.3 77.8,76.1 71.6,76.1 66.1,81.6 66.1,86.8 66.9,87.6 67.6,87.6 J2.1-5
  Bottom 0.15: C34.2 v81.6,71.5
C3.7  (via drill 0.3)
  Top 0.15: v84.4,71.5 78.4,77.5 72.3,77.5 68.7,81.1 68.7,86.7 69.5,87.5 70.04,87.5 J2.1-7
  Bottom 0.15: C59.1 v84.4,71.5
C3.8  (via drill 0.3)
  Top 0.15: v85.8,71.5 85,72.3 84.2,72.3 78.6,77.9 72.5,77.9 69.7,80.7 69.7,84.3 70.2,84.8 71.15,84.8 J2.1-8 72.5,86.07
  Bottom 0.15: C60.1 v85.8,71.5
C4.1  (via drill 0.3)
  Top 0.15: v81.4,8.5 82.3,8.5 92.8,19 92.8,62 87.8,67 87.8,71.5 77.5,81.8 77.5,82.8 77.5,83 77.5,88.61 J2.2-1
  Bottom 0.15: C23.2 v81.4,8.5
C4.2  (via drill 0.3)
  Top 0.15: v79.9,7.8 80,7.9 82.2,7.9 93.2,18.9 93.2,62.2 88.2,67.2 88.2,71.7 78.81,81.09 J2.2-2
  Bottom 0.15: v79.9,7.8 C24.2
C4.4  (via drill 0.3)
  Top 0.15: v84.6,7.8 84.6,8.8 94.5,18.7 94.5,62.9 89.4,68 89.4,72.1 81.35,80.15 J2.2-4
  Bottom 0.15: C31.2 v84.6,7.8
C4.5  (via drill 0.3)
  Top 0.15: v83.1,7.8 94.1,18.8 94.1,62.7 89,67.8 89,71.9 80.1,80.8 80.1,86.7 80.9,87.5 81.47,87.5 J2.2-5
  Bottom 0.15: C32.2 v83.1,7.8
C4.7  (via drill 0.3)
  Top 0.15: v86.2,9.2 95.4,18.4 95.4,63.6 90.2,68.8 90.2,72.4 82.6,80 82.6,86.8 83.2,87.4 83.91,87.4 J2.2-7
  Bottom 0.15: C61.1 v86.2,9.2
C4.8  (via drill 0.3)
  Top 0.15: J2.2-8 86.41,86.11 83.9,83.6 83.9,79.3 90.65,72.55 90.65,68.95 95.8,63.8 95.8,18.3 87.7,10.2 v87.7,9.2
  Bottom 0.15: C62.1 v87.7,9.2
CAPM1  (via drill 0.3)
  Top 0.15: U$1.CAPM(47) 14.4,54.35 | 14.4,54.35 12.95,54.35 11.2,56.1 11.2,64 13.2,66 v13.2,67 | v6.8,70 4.8,72 4.8,83.4 2.9,85.3 2.04,85.3 JP1.3 | U$1.CAPM(125) 26.1,42.8 v26,42.9 | v21.9,44 15.5,44 v15.4,43.9 | v14.4,48.6 14.4,54.35
  Bottom 0.15: v6.8,70 9.8,67 v13.2,67 | v26,42.9 25.7,43.2 22.7,43.2 v21.9,44 | v14.4,48.6 14.4,44.9 v15.4,43.9
CAPM2  (via drill 0.3)
  Top 0.15: U$2.CAPM(47) 14.2,34.35 | 14.2,34.35 12.05,34.35 9,37.4 9,63.7 10.9,65.6 v11.8,65.6 | v5.4,68.6 5.4,69.4 4,70.8 4,75.2 2.7,76.5 2.04,76.5 JP2.3 | U$2.CAPM(125) v25.9,22.8 | v21.5,23.8 v14.8,23.8 | v14.2,28.6 14.2,34.35
  Bottom 0.15: v5.4,68.6 8.4,65.6 v11.8,65.6 | v25.9,22.8 22.5,22.8 v21.5,23.8 | v14.8,23.8 14.8,28 v14.2,28.6
CAPM3  (via drill 0.3)
  Top 0.15: v89.1,64 89.1,62 90,61.1 90,54.8 86.2,51 | v93.7,69.4 95.3,71 95.3,83.4 97.24,85.34 JP3.3 | U$3.CAPM(47) 81.25,46.05 86.2,51 | U$3.CAPM(125) v73.95,57.6 | v84.25,56.5 78.25,56.5 v78.15,56.4 | v85.55,51.7 86.2,51.05 86.2,51
  Bottom 0.15: v89.1,64 93.7,68.6 v93.7,69.4 | v73.95,57.6 76.95,57.6 v78.15,56.4 | v84.25,56.5 84.25,53 v85.55,51.7
CAPM4  (via drill 0.3)
  Top 0.15: U$4.CAPM(47) 81.75,26.05 86.5,30.8 | v90.5,62.8 90.5,61.9 91.4,61 91.4,35.7 86.5,30.8 | v95.1,68.2 95.1,68.9 95.4,69.2 95.4,70 96.1,70.7 96.1,75.5 97.1,76.5 97.96,76.5 JP4.3 | U$4.CAPM(125) 73.8,37.6 v74,37.4 | v78.2,36.4 83.7,36.4 v84.2,36.9 | v85.6,31.7 86.5,30.8
  Bottom 0.15: v90.5,62.8 95.1,67.4 v95.1,68.2 | v74,37.4 74.1,37.3 77.3,37.3 v78.2,36.4 | v84.2,36.9 85.6,35.5 v85.6,31.7
CLK1+  (via drill 0.3)
  Top 0.15: U$1.CLK+(93) 21.15,47.65 20.9,47.4 v13,47.4
  Top 0.3: R49.2 18.7,66.95 v18.7,67.9
  Bottom 0.15: R39.2 v13,47.4 12.3,48.1 12.3,60.5 17.7,65.9 17.7,66.4 18,66.7 R45.1 18.65,66.9 R49.2
  Bottom 0.3: C20.1 18.7,69.05 v18.7,67.9 18.65,67.85 R45.1
CLK1-  (via drill 0.3)
  Top 0.15: U$1.CLK-(92) v13.65,47.95
  Top 0.3: R50.2 19.9,66.95 v19.9,67.9
  Bottom 0.15: R40.2 14.5,43.9 13.65,44.75 v13.65,47.95 12.7,48.9 12.7,60.4 18,65.7 19.7,65.7 20,66 20,66.65 R45.2
  Bottom 0.3: C19.1 19.9,68.95 v19.9,67.9 19.95,67.85 R45.2
CLK2+  (via drill 0.3)
  Top 0.15: U$2.CLK+(93) 21.05,27.65 20.8,27.4 v13,27.4 | R41.2 39.4,13.2 34.5,8.3 25.3,8.3 21.9,11.7 21.1,11.7 v20.2,12.6
  Top 0.3: 20.2,13.45 R51.2 20.3,12.7 v20.2,12.6
  Bottom 0.15: R39.1 13,40.1 12.3,39.4 12.3,28.1 v13,27.4 13.7,26.7 13.7,19.8 17.3,16.2 19.5,16.2 20.35,15.35 R46.1
  Bottom 0.3: R46.1 20.35,12.75 v20.2,12.6 20.1,12.5 C21.1
CLK2-  (via drill 0.3)
  Top 0.15: U$2.CLK-(92) 13.65,27.95 v13.6,28 | R42.2 48.6,14.7 47.5,13.6 39.2,13.6 34.3,8.7 25.5,8.7 v21.6,12.6
  Top 0.3: R52.2 21.6,13.45 v21.6,12.6
  Bottom 0.15: v13.6,28 12.7,28.9 12.7,39.2 14.5,41 R40.1 | v13.6,28 13.7,27.9 | v13.6,28 14.1,27.5 14.1,20 17.5,16.6 20.1,16.6 21.6,15.1 21.6,13.95 R46.2 | 21.65,12.65 v21.6,12.6
  Bottom 0.3: R46.2 21.65,12.65 | C22.1 v21.6,12.6
CLK3+  (via drill 0.3)
  Top 0.15: U$3.CLK+(93) 78.75,52.75 79.1,53.1 v86.9,53.1 86,53.1
  Top 0.3: R55.2 80,67.9 v79.9,68
  Bottom 0.15: R43.1 86.7,40.2 87.7,41.2 87.7,52.3 v86.9,53.1 85.3,54.7 85.3,61.4 80.8,65.9 80.8,66.6 80.4,67 R48.1
  Bottom 0.3: C25.1 v79.9,68 79.85,67.95 R48.1
CLK3-  (via drill 0.3)
  Top 0.15: U$3.CLK-(92) 86.25,52.45 v86.3,52.5
  Top 0.3: v78.5,68 R56.2
  Bottom 0.15: R44.1 85.4,39.4 87.3,41.3 87.3,51.5 v86.3,52.5 84.9,53.9 84.9,61.2 80.6,65.5 79.1,65.5 78.5,66.1 R56.2 R48.2
  Bottom 0.3: C26.1 78.5,69.05 v78.5,68 78.5,67.05 R48.2
CLK4+  (via drill 0.3)
  Top 0.15: U$4.CLK+(93) 78.75,32.75 79.1,33.1 v86.9,33.1 | R41.1 59.9,13.2 64.8,8.3 76.4,8.3 79.8,11.7 80.6,11.7 v81.4,12.5
  Top 0.3: R53.2 v81.4,12.5
  Bottom 0.15: R43.2 86.9,37.15 v86.9,33.1 88.1,31.9 88.1,19.5 85,16.4 82.7,16.4 81.35,15.05 R47.1
  Bottom 0.3: C23.1 v81.4,12.5 81.4,13.75 R47.1
CLK4-  (via drill 0.3)
  Top 0.15: U$4.CLK-(92) 86.25,32.45 v86.3,32.5 | R42.1 51.5,14.7 52.6,13.6 60.1,13.6 65,8.7 76.2,8.7 v80,12.5
  Top 0.3: v80,12.5 R54.2
  Bottom 0.15: R44.2 85.4,36.7 86.3,35.8 v86.3,32.5 87.7,31.1 87.7,19.7 84.8,16.8 82.5,16.8 80.2,14.5 80.2,13.95 R47.2
  Bottom 0.3: C24.1 80,11.45 v80,12.5 80,13.75 R47.2
CMD1+  (via drill 0.3)
  Top 0.15: U$1.CMD+(95) 21.55,47.05 20.7,46.2 v11.8,46.2
  Top 0.3: v15.5,67.9 R67.2
  Bottom 0.15: R57.2 10,43.9 10.4,44.3 11.2,44.3 11.8,44.9 v11.8,46.2 11,47 11,61.6 15.45,66.05 R63.1
  Bottom 0.3: C27.1 15.5,69.05 v15.5,67.9 15.45,67.85 R63.1
CMD1-  (via drill 0.3)
  Top 0.15: U$1.CMD-(94) 21.35,47.35 20.8,46.8 v12.4,46.8
  Top 0.3: R68.2 v16.8,67.9
  Bottom 0.15: R58.2 11.5,43.9 12.4,44.8 v12.4,46.8 11.4,47.8 11.4,61.5 15.3,65.4 16.3,65.4 16.8,65.9 16.8,66.65 R63.2
  Bottom 0.3: C28.1 16.8,69.05 v16.8,67.9 16.75,67.85 R63.2
CMD2+  (via drill 0.3, 0.3 pad 0.7)
  Top 0.15: U$2.CMD+(95) 21.45,27.05 20.6,26.2 v11.8,26.2 | R59.2 48.5,10 47.3,11.2 39.4,11.2 35.3,7.1 24.5,7.1 21.2,10.4 19,10.4 v16.8,12.6
  Top 0.3: 17.1,13.45 R69.2 v16.8,12.6
  Bottom 0.15: R57.1 10,40.7 11.1,39.6 11.1,26.9 v11.8,26.2 12.5,25.5 12.5,19.2 16.95,14.75 R64.1
  Bottom 0.3: C29.1 v16.8,12.6 16.95,12.75 R64.1
CMD2-  (via drill 0.3)
  Top 0.15: U$2.CMD-(94) 21.25,27.35 20.7,26.8 v12.4,26.8 | R60.2 39.1,11.6 35,7.5 24.7,7.5 21.4,10.8 20.3,10.8 18.5,12.6 v18.4,12.6
  Top 0.3: 18.6,13.35 R70.2 v18.4,12.6
  Bottom 0.15: v12.4,26.8 11.5,27.7 R58.1 | v12.4,26.8 12.5,26.7 | v12.4,26.8 12.9,26.3 12.9,19.4 17,15.3 17.7,15.3 18.3,14.7 18.3,13.95 R64.2
  Bottom 0.3: R64.2 18.25,12.75 v18.4,12.6 C30.1
CMD3+  (via drill 0.3)
  Top 0.15: U$3.CMD+(95) 78.35,53.35 79.3,54.3 v88.1,54.3
  Top 0.3: R73.2 83.1,67.8 v82.9,68
  Bottom 0.15: R61.1 89.9,39.4 88.8,40.5 88.8,53.6 v88.1,54.3 86.6,55.8 86.6,61.9 83,65.5 83,66.95 R66.1 82.9,66.95
  Bottom 0.3: C33.1 83,68.1 v82.9,68 82.9,67.05 R66.1
CMD3-  (via drill 0.3)
  Top 0.15: U$3.CMD-(94) 78.55,53.05 79.2,53.7 v87.5,53.7
  Top 0.3: R74.2 v81.6,68
  Bottom 0.15: R62.1 88.4,52.8 v87.5,53.7 86.25,54.95 86.25,61.65 81.65,66.25 R66.2
  Bottom 0.3: C34.1 v81.6,68 81.6,67.05 R66.2
CMD4+  (via drill 0.3)
  Top 0.15: U$4.CMD+(95) 78.35,33.35 79.3,34.3 v88.1,34.3 | R59.1 51.2,10 52.4,11.2 60.1,11.2 64.2,7.1 76.9,7.1 80.3,10.5 82.5,10.5 v84.5,12.5
  Top 0.3: R71.2 v84.5,12.5
  Bottom 0.15: R61.2 89.9,36.7 89.6,36.4 89,36.4 88.1,35.5 v88.1,34.3 89.3,33.1 89.3,18.9 85.5,15.1 84.8,15.1 84.35,14.65 R65.1
  Bottom 0.3: R65.1 84.5,13.65 v84.5,12.5 84.5,11.45 C31.1
CMD4-  (via drill 0.3)
  Top 0.15: U$4.CMD-(94) 78.55,33.05 79.2,33.7 v87.5,33.7 | R60.1 60.3,11.6 64.4,7.5 76.7,7.5 80.1,10.9 81.5,10.9 v83.1,12.5
  Top 0.3: v83.1,12.5 R72.2
  Bottom 0.15: R62.2 88.4,36.7 87.5,35.8 v87.5,33.7 88.9,32.3 88.9,19.1 85.3,15.5 83.8,15.5 83.1,14.8 83.1,13.85 R65.2
  Bottom 0.3: R65.2 83.1,13.75 v83.1,12.5 C32.1
DOB1+  (via drill 0.3)
  Top 0.15: U$1.DOB+(103) 21.75,46.25 21.1,45.6 v11.2,45.6
  Bottom 0.15: v11.2,45.6 10.2,46.6 10.2,62 14.5,66.3 14.5,67.6 13.6,68.5 C55.2
DOB1-  (via drill 0.3)
  Top 0.15: U$1.DOB-(104) 21.95,45.95 21,45 v10.6,45
  Bottom 0.15: v10.6,45 9.8,45.8 9.8,62.1 14.1,66.4 14.1,67.4 13.2,68.3 12.5,68.3 12.2,68.6 C56.2
DOB2+  (via drill 0.3)
  Top 0.15: U$2.DOB+(103) 21.75,26.25 21.1,25.6 v11.2,25.6
  Bottom 0.15: v11.2,25.6 11.7,25.1 11.7,18.9 15.8,14.8 15.8,12.8 15.2,12.2 C57.2
DOB2-  (via drill 0.3)
  Top 0.15: U$2.DOB-(104) 21.95,25.95 21,25 v10.6,25
  Bottom 0.15: v10.6,25 11.3,24.3 11.3,18.7 15.4,14.6 15.4,13.1 14.6,12.3 14,12.3 13.7,12 C58.2
DOB3+  (via drill 0.3)
  Top 0.15: U$3.DOB+(103) 78.25,54.15 79,54.9 v88.7,54.9
  Bottom 0.15: v88.7,54.9 87.45,56.15 87.45,62.3 83.8,65.95 83.8,67.9 84.4,68.5 C59.2
DOB3-  (via drill 0.3)
  Top 0.15: U$3.DOB-(104) 78.05,54.45 79.1,55.5 v89.3,55.5
  Bottom 0.15: v89.3,55.5 87.9,56.9 87.9,62.4 84.2,66.1 84.2,67.7 84.8,68.3 85.5,68.3 85.8,68.6 C60.2
DOB4+  (via drill 0.3)
  Top 0.15: U$4.DOB+(103) 78.25,34.15 79,34.9 v88.7,34.9
  Bottom 0.15: v88.7,34.9 90,33.6 90,18.4 86.2,14.6 C61.2
DOB4-  (via drill 0.3)
  Top 0.15: U$4.DOB-(104) 78.05,34.45 79.1,35.5 v89.3,35.5
  Bottom 0.15: v89.3,35.5 90.4,34.4 90.4,18.3 87.7,15.6 C62.2
GND  (via drill 0.3, 0.3 pad 0.7, 0.9, 1 pad 1.78)
  Top 0.2: R100.4 R100.3 R100.2 | R3.4 R3.3 R3.2 R3.1 25.74,61.86 v25.7,61.9 | R4.1 R4.2 R4.3 | R4.3 v26.5,19.9 | R4.3 R4.4 | R100.2 25.8,41.4 v25.8,41.5 | R100.2 R100.1 | R30.1 R30.2 R30.3 R30.4 74.16,59.86 v74.2,59.9 | R31.2 74.15,38.95 v74.2,38.9 | R31.1 R31.2 | R31.2 R31.3 R31.4 | R32.4 R32.3 R32.2 R32.1 74.2,18.54 v74.2,18.6
  Top 0.3: 20.4,14.95 R51.1 | R67.1 15.5,64.05 C51.1 | 27.9,59.8 v28.1,59.6 28.2,59.7 | 27.9,42.6 v28.1,42.8 28.2,42.7 | 27.9,39.8 v28.1,39.6 28.2,39.7 | C54.1 83.05,65.6 R73.1 | v71.9,48.8 U$3.GND | U$4.GND v71.9,28.8 | U$2.GND v28.1,30.8 | C13.2 C14.2 | C40.2 78.25,44.3
  Top 0.4: C5.2 C6.2
  Top 0.5: R10.1 v22.8,56.5 | R19.1 v22.8,36.6 | R37.1 v77.1,23.8 | C53.1 v78.6,12.5 | v18.6,64.8 R49.1 | R28.1 v77.1,43.8 | R20.1 v22.8,38 | R92.1 v22.8,39.4 | R90.1 v22.8,59.3 | R11.1 v22.8,57.9 | R29.1 v77.1,42.4 | R38.1 v77.1,22.4 | R93.1 v77.1,21 | 20.4,14.95 20.4,15.5 20.9,16 v21.7,16 | C52.1 v23.2,12.6 | R69.1 15.15,14.85 v14.6,14.3 | C2.2 v57.6,69.3 | C1.2 v35.9,69.3 | R53.1 81.4,15.4 81,15.8 v80.5,15.8 | C41.2 v22.8,40.6 | C38.2 v22.9,42.3 | v15.8,62.6 15.55,62.85 C51.1 | C50.2 v77.1,19.8 | C46.2 v77.1,39.8 | C49.2 v77.1,38.1 | R55.1 v80,64.8 | C54.1 83.05,63.55 v82.3,62.8 | C37.2 v22.9,60.6 | v28.1,50.8 U$1.GND | R85.1 v54.7,90.6 | R71.1 v84.5,17.5 | C3.2 v22.8,55.4 | C4.2 v22.9,53.1 | C6.2 v22.9,48.8 | R102.1 v19,60.8 | C35.2 20.65,55.85 v20.6,55.9 | C42.2 v22.9,21.6 | C44.2 v22.9,24 | C43.2 20.65,36.05 v20.6,36.1 | C7.2 v22.8,35.4 | R104.1 v18.9,41 R15.1 | v22.9,28.8 C10.2 C9.2 | C8.2 v22.9,32.8 | R76.1 v18.9,21 | C36.2 v22.9,44 | C45.2 v77.1,58.3 | C14.2 v77.2,51.7 | C12.2 v77.1,47.4 | C15.2 v77.1,25 | C16.2 v77.2,27.4 | C18.2 v77.2,31.6 | C17.2 v77.2,30.2 | R77.1 v80.7,59.4 | C39.2 v77.1,56.4 | C11.2 v77.1,45 | R91.1 v77.1,41 | C48.2 79.05,24.45 v79.1,24.5 | R88.1 v80.7,19.5 | C47.2 v77.1,36.4 | 78.25,44.3 v79.1,44.3 | R86.1 v81,39.5 R83.1
  Top 1: C63.- v61.6,65.1 | C64.- v61.2,77.7
  other vias: 52.55,97.55 52.55,92.45 47.45,97.55 47.45,92.45 28.1,44.4 28.1,43.6 28.1,45.2 28.1,46 28.1,46.8 28.1,47.6 28.1,48.4 28.1,51.6 28.1,50 28.1,49.2 28.1,58.8 28.1,58 28.1,57.2 28.1,56.4 28.1,55.6 28.1,54.8 28.1,54 28.1,53.2 28.1,52.4 28.1,24.4 28.1,23.6 28.1,25.2 28.1,26 28.1,26.8 28.1,27.6 28.1,28.4 28.1,31.6 28.1,30 28.1,29.2 28.1,38.8 28.1,38 28.1,37.2 28.1,36.4 28.1,35.6 28.1,34.8 28.1,34 28.1,33.2 28.1,32.4 71.9,42.4 71.9,41.6 71.9,43.2 71.9,44 71.9,44.8 71.9,45.6 71.9,46.4 71.9,49.6 71.9,48 71.9,47.2 71.9,56.8 71.9,56 71.9,55.2 71.9,54.4 71.9,53.6 71.9,52.8 71.9,52 71.9,51.2 71.9,50.4 71.9,22.4 71.9,21.6 71.9,23.2 71.9,24 71.9,24.8 71.9,25.6 71.9,26.4 71.9,29.6 71.9,28 71.9,27.2 71.9,36.8 71.9,36 71.9,35.2 71.9,34.4 71.9,33.6 71.9,32.8 71.9,32 71.9,31.2 71.9,30.4 28.1,22.8 71.9,40.8 71.9,57.6 71.9,37.6 71.9,20.8
  pour Bottom: 0.1,99.9 0.1,0.1 99.9,0.1 99.9,99.9 48.5,99.9 48.5,89.2 50,87.7 50,78 48.5,76.5 41,76.5 39.5,78 39.5,87.7 41,89.2 48.4,89.2 48.4,99.9
HITOR  (via drill 0.3, 1 pad 1.78)
  Top 0.15: R81.2 78.2,55.2 78.9,55.9 88.6,55.9 v89.3,56.6 89.3,60.9 87.1,63.1 87.1,71.3 75.6,82.8 75.6,89.1 74.1,90.6 v64.8,90.6 | R82.2 78.2,35.2 79,36 84.9,36 85.2,36.3 90.4,36.3 v90.5,36.2 | R80.2 21.8,25.2 21.1,24.5 14.1,24.5 13.5,23.9 v9.5,23.9 9.5,17.5 17.5,9.5 20.7,9.5 24,6.2 77.1,6.2 80.7,9.8 82.9,9.8 92,18.9 v92,34.7 | v62.2,90.6 R85.2 | R79.2 21.9,45.2 21.3,44.6 14.6,44.6 10.5,40.5 v10.5,39.2
  Top 0.3: R85.2 57.65,91.35 57.1,91.9 55.4,91.9 53.8,93.5 v53.8,95
  Bottom 0.15: v64.8,90.6 v62.2,90.6 | v89.3,56.6 90.1,55.8 90.1,40.3 90.9,39.5 90.9,36.6 v90.5,36.2 v92,34.7 | v10.5,39.2 10.5,26.8 9.5,25.8 v9.5,23.9
  Bottom 0.3: v50,95 v53.8,95
LDO1.1
  Top 0.3: U$6.P$4 28.95,41.45 28.75,41.65 U$1.VDDA 28.75,61.25 29,61.5 U$5.P$4
LDO1.2
  Top 0.3: U$5.P$6 U$5.P$8 29.2,60.3 29.2,42.15 U$6.P$2
LDO2.1
  Top 0.3: U$6.P$6 28.95,40.95 28.75,40.75 U$2.VDDA 28.75,21.05 28.9,20.9 U$7.P$6
LDO2.2
  Top 0.3: U$7.P$4 U$7.P$2 29.2,22.1 29.2,40.25 U$6.P$8
LDO3.1
  Top 0.3: U$9.P$6 71,39.4 71.25,39.65 U$3.VDDA 71.25,59.25 71,59.5 U$10.P$6
LDO3.2
  Top 0.3: U$10.P$4 U$10.P$2 70.8,58.3 70.8,40.1 U$9.P$8
LDO4.1
  Top 0.3: U$9.P$4 71,38.9 71.25,38.65 U$4.VDDA 71.25,19.05 71.1,18.9 U$8.P$4
LDO4.2
  Top 0.3: U$9.P$2 70.8,38.2 70.8,20.1 U$8.P$8 U$8.P$6
N$1
  Top 0.5: BACKPLANE.TP 50.02,64.72 R2.2 C2.1
N$2
  Top 0.5: C1.1 43.68,69.3 R1.2 47.16,69.28 R2.1
N$3  (via drill 0.3)
  Top 0.15: v25.8,89.5 23.4,91.9 13.13,91.9 9.6,88.37 9.6,86.1 8.8,85.3 7.03,85.3 JP13.2 | U$17.P$1 35.8,63.3 36,63.5 36,64 35.8,64.2 35.2,64.2 34.8,64.6 34.8,73.4 30,78.2 v29,78.2
  Bottom 0.15: v25.8,89.5 25.8,86.4 28.6,83.6 28.6,78.6 v29,78.2
N$4
  Top 0.15: U$1.RESET1(45) 26.25,54.95 25.9,55.3 25.15,55.3 C3.1
N$5
  Top 0.15: U$1.RESET2(56) 25.15,53.2 C4.1
N$6
  Top 0.15: U$1.RESET3(88) 26.55,48.65 26.5,48.7 26.5,49.1 25.6,50 25.25,50 C5.1
N$7
  Top 0.15: U$1.RESET4(89) 26.25,48.35 25.9,48.7 25.15,48.7 C6.1
N$8
  Top 0.15: U$1.GA0(67) 26.5,51.7 26.1,52.1 21.95,52.1 R7.1
N$9
  Top 0.15: U$1.GA1(68) 26.35,51.35 25.9,51.8 23,51.8 22.4,51.2 21.95,51.2 R8.1
N$10
  Top 0.15: U$1.GA2(69) 26.2,51 25.7,51.5 23.4,51.5 22.7,50.8 22.7,49.9 22.5,49.7 R9.1
N$11
  Top 0.15: U$1.IREF(33,34) 25.1,56.55 R10.2
N$12
  Top 0.15: U$1.VTHR(24,16) 26.1,58.3 25.7,57.9 R11.2
N$13
  Top 0.15: R79.1 25.9,45.2 26.25,45.55 U$1.HITOR(105)
N$14
  Top 0.15: U$2.GA0(67) 26.4,31.7 26.1,32 22.7,32 22.3,32.4 21.75,32.4 R16.1 21.85,32.3
N$15
  Top 0.15: U$2.GA1(68) 26.25,31.35 25.9,31.7 23.2,31.7 22.7,31.2 R17.1 21.75,31.3
N$16
  Top 0.15: U$2.GA2(69) 26.1,31 25.7,31.4 23.5,31.4 22.9,30.8 22.9,30.3 22.4,29.8 R18.1 21.85,30
N$17
  Top 0.15: U$2.RESET1(45) 26.05,34.95 25.7,35.3 25.15,35.3 C7.1
N$18
  Top 0.15: U$2.RESET2(56) 26.5,33.2 26.1,32.8 C8.1
N$19
  Top 0.15: U$2.RESET3(88) 26.55,28.65 26.5,28.7 26.5,29.1 25.7,29.9 25.35,29.9 C9.1
N$20
  Top 0.15: U$2.RESET4(89) 26.25,28.35 25.9,28.7 25.25,28.7 25.15,28.8 C10.1
N$21
  Top 0.15: U$2.HITOR(105) 26.45,25.55 26.1,25.2 R80.1
N$22
  Top 0.15: U$3.HITOR(105) 73.75,54.85 74.1,55.2 R81.1
N$23
  Top 0.15: U$4.HITOR(105) 73.85,34.85 74.2,35.2 R82.1
N$24
  Top 0.15: U$1.TDAC(11) 25.05,59.15 R90.2
N$25
  Top 0.15: U$2.IREF(33,34) 25.1,36.55 R19.2
N$26
  Top 0.15: U$2.VTHR(24,16) 26,38.3 25.7,38 R20.2
N$27
  Top 0.15: U$3.TDAC(11) 74.95,41.25 R91.2
N$28
  Top 0.15: 25.15,39.3 R92.2 25.3,39.15 U$2.TDAC(11)
N$29
  Top 0.15: 74.75,21.3 R93.2 74.3,21 74.05,21.25 U$4.TDAC(11)
N$30  (via drill 0.3)
  Top 0.15: v28.2,77.3 30.3,77.3 34.4,73.2 34.4,63.9 34.5,63.8 U$17.P$2 | v24.6,89.5 22.6,91.5 13.3,91.5 10,88.2 10,83.6 9.1,82.7 7.03,82.7 JP13.1
  Bottom 0.15: v28.2,77.3 28.2,83.5 25.4,86.3 25.4,88.7 v24.6,89.5
N$31
  Top 0.15: U$18.P$2 65.4,63.8 65.4,77 61.8,80.6 61.8,88.7 64.6,91.5 86.8,91.5 89.5,88.8 89.5,84.1 90.77,82.83 JP14.1
N$32
  Top 0.15: U$18.P$1 64.2,63.3 64,63.5 64,64 64.3,64.3 64.7,64.3 65,64.6 65,76.9 61.4,80.5 61.4,88.8 64.5,91.9 87.1,91.9 90,89 90,86 90.6,85.4 92.97,85.4 JP14.2
N$33
  Top 0.15: R3.8 27.66,61.86 27.8,62 U$5.P$1
N$34
  Top 0.5: X1.1 R1.1
N$35
  Top 0.15: R12.1 21.65,22.5 22.5,22.5 22.8,22.8 25,22.8 25.6,23.4 26.3,23.4 26.5,23.2 U$2.REXT1(120)
N$38
  Top 0.15: R3.5 27.66,60.64 27.8,60.5 U$5.P$7
N$39
  Top 0.15: R3.7 28.15,61.45 U$5.P$3
N$40
  Top 0.15: R3.6 28.15,61.05 U$5.P$5
N$41
  Top 0.15: U$6.P$1 27.85,41.95 27.7,41.8 R100.8
N$42
  Top 0.15: U$6.P$3 28.15,41.4 R100.7
N$43
  Top 0.15: U$6.P$5 28.15,41 R100.6
N$44
  Top 0.15: R100.5 27.71,40.59 27.85,40.45 U$6.P$7
N$45
  Top 0.15: R4.8 27.66,21.76 27.8,21.9 U$7.P$1
N$46  (via drill 0.3)
  Top 0.15: U$21.P$2 25.1,17.1 24.7,16.7 24.7,11.6 v24.3,11.2 | v22.7,5.1 11.9,5.1 9.7,7.3 9.7,11.2 4.2,16.7 4.2,65.7 7.9,69.4 7.9,74.8 9,75.9 9,78.1 7.9,79.2 7.07,79.2 JP9.1
  Bottom 0.15: v24.3,11.2 24.3,6.7 v22.7,5.1
N$47  (via drill 0.3)
  Top 0.15: U$21.P$1 25.3,16.6 25.1,16.4 v25.1,10.4 | v23.3,4.4 22.3,4.4 22,4.7 11.7,4.7 9.3,7.1 9.3,11.1 3.8,16.6 3.8,65.9 7.5,69.6 7.5,76.23 JP9.2
  Bottom 0.15: v25.1,10.4 25.1,6.2 v23.3,4.4
N$48  (via drill 0.3)
  Top 0.15: U$22.P$2 75.2,17.1 76.1,16.2 76.1,10.5 v76.5,10.1 | v78.9,6.7 86.9,6.7 96.8,16.6 96.8,64.2 92.6,68.4 92.6,74.3 91,75.9 91,78.1 92.1,79.2 92.93,79.2 JP10.1
  Bottom 0.15: v76.5,10.1 76.5,8.4 78.2,6.7 v78.9,6.7
N$49  (via drill 0.3)
  Top 0.15: U$22.P$1 75,16.6 75.7,15.9 v75.7,9.5 | v78.2,6 86.8,6 97.2,16.4 97.2,64.5 93,68.7 JP10.2
  Bottom 0.15: v75.7,9.5 75.7,8.5 v78.2,6
N$50
  Top 0.15: U$3.GA2(69) 73.9,49.4 74.3,49 76.5,49 77.8,50.3 78.05,50.3 R27.1
N$51
  Top 0.15: 21.65,42.6 R5.1 22.35,42.65 22.7,43 25.3,43 25.5,43.2 25.8,43.5 26.2,43.5 26.5,43.2 U$1.REXT1(120)
N$52
  Top 0.15: U$1.REXT2(B7) 26,58.8 25.8,58.6 21.65,58.6 R6.1
N$53
  Top 0.15: R4.7 28.15,21.35 U$7.P$3
N$54
  Top 0.15: R4.6 28.15,20.95 U$7.P$5
N$55
  Top 0.15: R4.5 27.66,20.54 27.8,20.4 U$7.P$7
N$56
  Top 0.15: U$3.IREF(33,34) 74.9,43.85 R28.2
N$57
  Top 0.15: U$3.GA1(68) 73.75,49.05 74.2,48.6 77.3,48.6 77.8,49.1 78.25,49.1 R26.1
N$58
  Top 0.15: U$3.GA0(67) 73.6,48.7 74.1,48.2 77.4,48.2 77.6,48 78.15,48 R25.1
N$59
  Top 0.15: U$3.RESET1(45) 73.95,45.45 74.3,45.1 74.85,45.1 C11.1
N$60
  Top 0.15: U$3.RESET2(56) 74.85,47.2 C12.1
N$61
  Top 0.15: U$3.RESET3(88) 73.45,51.75 73.5,51.7 73.5,51.3 74.1,50.7 74.65,50.7 C13.1
N$62
  Top 0.15: U$3.RESET4(89) 73.85,52.05 74.1,51.8 74.85,51.8 C14.1
N$63
  Top 0.15: U$2.REXT2(B7) 25.9,38.8 25.8,38.7 21.75,38.7 R13.1
N$64
  Top 0.15: U$3.VTHR(24,16) 73.9,42.1 74.2,42.4 R29.2
N$65
  Top 0.15: R21.1 78.05,57.8 77.5,57.8 77.2,57.5 74.65,57.5 74.2,57.05 73.7,57.05 73.55,57.2 U$3.REXT1(120)
N$66
  Top 0.15: U$3.REXT2(B7) 74.1,41.6 74.2,41.7 78.15,41.7 R22.1
N$67
  Top 0.15: R23.1 78.05,37.6 77.4,37.6 77.2,37.4 74.8,37.4 74.25,36.85 73.75,36.85 73.4,37.2 U$4.REXT1(120)
N$68
  Top 0.15: U$4.REXT2(B7) 74,21.6 74.1,21.7 78.05,21.7 R24.1
N$69
  Top 0.15: R30.5 72.34,59.86 72.2,60 U$10.P$7
N$70
  Top 0.15: R30.8 72.34,58.64 72.2,58.5 U$10.P$1
N$71
  Top 0.15: R30.6 71.85,59.45 U$10.P$5
N$72
  Top 0.15: R30.7 71.85,59.05 U$10.P$3
N$73
  Top 0.15: R34.1 78.15,27.7 77.8,27.7 77.2,28.3 73.9,28.3 73.5,28.7 U$4.GA0(67)
N$74
  Top 0.15: R35.1 78.15,28.6 74.1,28.6 73.65,29.05 U$4.GA1(68)
N$75
  Top 0.15: R36.1 78.05,29.8 77.8,29.8 76.9,28.9 74.3,28.9 73.8,29.4 U$4.GA2(69)
N$76
  Top 0.15: U$4.RESET1(45) 73.75,25.45 74.2,25 C15.1
N$77
  Top 0.15: U$4.RESET2(56) 74.75,27.2 C16.1
N$78
  Top 0.15: U$4.RESET3(88) 73.45,31.75 73.5,31.7 73.5,31.3 74.4,30.4 74.75,30.4 C17.1
N$79
  Top 0.15: U$4.RESET4(89) 73.75,32.05 74.1,31.7 74.85,31.7 C18.1
N$80
  Top 0.15: U$4.IREF(33,34) 74.8,23.85 R37.2
N$81
  Top 0.15: U$4.VTHR(24,16) 73.9,22.1 74.1,22.3 74.85,22.3 R38.2
N$82
  Top 0.15: R31.6 71.85,39.35 U$9.P$5
N$83
  Top 0.15: R31.5 72.34,39.76 72.2,39.9 U$9.P$7
N$84
  Top 0.15: R31.8 72.34,38.54 72.2,38.4 U$9.P$1
N$85
  Top 0.15: R31.7 71.85,38.95 U$9.P$3
N$86
  Top 0.15: R32.5 72.34,19.76 72.2,19.9 U$8.P$7
N$87
  Top 0.15: R32.6 71.85,19.35 U$8.P$5
N$88
  Top 0.15: R32.7 71.85,18.95 U$8.P$3
N$89
  Top 0.15: R32.8 72.34,18.54 72.2,18.4 U$8.P$1
NTC1+
  Top 0.15: J1.2-3 31.33,89.9 36.6,89.9 38,88.5 38,84.4 36.7,83.1 35.9,83.1 34.47,81.67 JP5.1
NTC1-
  Top 0.15: J1.2-6 35.18,87.4 36.8,87.4 37.6,86.6 37.6,84.7 36.5,83.6 34.1,83.6 31.9,81.4 31.9,79.63 JP5.2
NTC2+
  Top 0.15: J1.1-3 17.36,89.9 23,89.9 24.5,88.4 24.5,84.33 23.97,83.8 JP6.1
NTC2-
  Top 0.15: J1.1-6 21.21,87.4 23.3,87.4 24,86.7 24,85.4 23.4,84.8 22.4,84.8 21.43,83.83 JP6.2
NTC3+
  Top 0.15: J2.1-3 67.46,90 72.3,90 74.1,88.2 74.1,81.77 JP7.1
NTC3-
  Top 0.15: J2.1-6 71.21,87.4 73,87.4 73.6,86.8 73.6,85.2 73.1,84.7 72,84.7 71.6,84.3 71.6,81.73 JP7.2
NTC4+
  Top 0.15: J2.2-3 81.53,90.1 86.5,90.1 88.3,88.3 88.3,81.77 JP8.1
NTC4-
  Top 0.15: J2.2-6 85.18,87.4 87.1,87.4 87.8,86.7 87.8,85.4 87.2,84.8 86.3,84.8 85.8,84.3 85.8,81.73 JP8.2
REF1.1
  Top 0.15: R103.1 20.65,43.3 24.8,43.3 24.9,43.4 24.9,43.85 C36.1 | C36.1 25,44 | U$1.VREF1(119) 26.6,43.5 26.3,43.8 25.25,43.8 C36.1
  Top 0.3: R104.2 R103.1
REF1.2
  Top 0.15: U$1.VREF2(B8) 26.4,57.9 25.7,57.2 21.65,57.2 C35.1
  Top 0.3: R102.2 R101.1 20.3,57.6 20.7,57.2 21.65,57.2
REF2.1
  Top 0.15: R75.1 20.45,23.2 24.8,23.2 25,23.4 25,23.95 C44.1 25.35,23.7 26.4,23.7 26.6,23.5 U$2.VREF1(119)
  Top 0.3: R75.1 R76.2
REF2.2
  Top 0.15: U$2.VREF2(B8) 26.3,37.9 25.7,37.3 21.85,37.3 C43.1
  Top 0.3: R15.2 R14.1 20.3,37.8 20.75,37.35 C43.1
REF3.1
  Top 0.15: R77.2 R33.1 79.4,57.2 75.25,57.2 75.05,57 75.05,56.5 C39.1 74.7,56.65 73.7,56.65 73.45,56.9 U$3.VREF1(119)
REF3.2
  Top 0.15: U$3.VREF2(B8) 73.7,42.5 74.3,43.1 78.1,43.1 C40.1
  Top 0.3: R83.2 R78.1 79.6,42.7 79.25,43.05 C40.1
REF4.1
  Top 0.15: C47.1 75,36.45 | R84.1 79.45,37.1 75.2,37.1 75.1,37 75.1,36.55 C47.1 | U$4.VREF1(119) 73.3,36.9 73.65,36.55 74.8,36.55 C47.1
  Top 0.3: R84.1 R86.2
REF4.2
  Top 0.15: U$4.VREF2(B8) 73.7,22.5 74.3,23.1 78.05,23.1 C48.1
  Top 0.3: C48.1 78.95,23.15 79.4,22.7 R87.1 R88.2
VDDA  (via drill 0.3 pad 0.7)
  Top 0.3: 24.7,62.6 28.8,62.6 U$5.P$2 | U$10.P$8 71.4,60.8 72.7,60.8
  Top 1: v31,72.3 v30.2,72.3 v29.4,72.3 v28.6,72.3 v27.8,72.3 24.9,69.4 24.9,66.3 23.9,65.3 23.9,63 24.3,62.6 24.7,62.6 | v68.7,72.3 v69.5,72.3 v70.3,72.3 v71.1,72.3 v71.9,72.3 74.6,69.6 74.6,65.8 75.8,64.6 75.8,63 73.6,60.8 72.7,60.8 | X1.3 52.1,76.9 56.7,72.3 v60,72.3 | v61.6,72.3 v62.4,72.3 v63.2,72.3 | v61.6,72.3 v60.8,72.3 v60,72.3 | 58.8,72.3 v60,72.3 | C63.+ v61.6,72.3
  Bottom 1: v27.8,72.3 v63.2,72.3 v68.7,72.3 v71.9,72.3
VDDD  (via drill 0.3 pad 0.7)
  Top 0.15: 72.55,29.9 U$4.VDDD | 27.45,30.5 27.45,30.2
  Top 0.3: U$3.VDDD 72.55,46.5 | 72.55,46.5 72.55,40.6 73.6,40.6 74.4,39.8 C46.1 74.95,39 | R27.2 R26.2 R25.2 79.65,46.95 79.2,46.5 72.55,46.5 | U$3.VDDD 72.55,49.8 | R54.1 C53.2 78.6,16.6 | R72.1 83.1,15.8 82.3,16.6 78.6,16.6 | 72.55,29.9 72.55,38.1 C49.1 74.95,39 | R50.1 20.05,65.6 20.05,64.85 | 27.45,33.8 U$2.VDDD 27.45,30.2 27.45,22.2 26.1,22.2 25.8,21.9 25.15,21.9 C42.1 25.05,20.5 | 27.45,33.8 27.45,39.8 26.4,39.8 25.65,40.55 25.1,40.55 C41.1 25.05,41.4 | 21.65,14.9 R52.1 C52.2 23.2,17.3 | R70.1 18.4,16.2 19.5,17.3 23.2,17.3 | 27.45,53.8 U$1.VDDD 27.45,42.2 25.15,42.2 C38.1 25.05,41.4 | 27.45,53.8 27.45,59.8 26.35,59.8 25.75,60.4 25.05,60.4 C37.1 | C51.2 16.8,64.05 R68.1 | C51.2 19.2,64 20.05,64.85 | 16.8,63.95 C51.2 | U$3.VDDD 72.55,58.25 74.9,58.25 C45.1 75.1,58.45 75.1,59.1 75.3,59.3 | 20.05,64.85 20.65,64.25 20.75,64.25 | R74.1 81.75,65.5 C54.2 81.65,64 78.5,64 | 78.7,65.45 R56.1 78.4,65.55 78.5,65.45 78.5,64 | 20.4,29.75 R18.2 R17.2 R16.2 20.35,33.25 20.9,33.8 27.45,33.8 | 23.2,17.3 25.05,19.15 25.05,20.5 | 79.7,30.15 R36.2 R35.2 R34.2 79.65,26.85 79.3,26.5 72.55,26.5 | 78.5,64 77.1,64 | U$4.VDDD 72.55,26.5 | 72.55,26.5 72.55,20.6 | 72.55,20.6 72.55,20.45 | R9.2 R8.2 R7.2 20.45,53.35 21,53.9 27.35,53.9 27.45,53.8 | 21.6,61.65 R6.2 R101.2 | R75.2 20.3,20.9 20.7,20.5 21.6,20.5 | 21.6,20.5 25.05,20.5 | R12.2 21.6,20.5 | R103.2 R14.2 R13.2 R5.2 21.6,41.4 25.05,41.4 | C50.1 74.4,19.8 73.6,20.6 72.55,20.6 | C50.1 74.95,18.75 | 75.3,60 75.3,59.3 | 75.3,59.3 77.95,59.3 R21.2 79.25,59.25 79.4,59.1 R33.2 | 78.6,16.6 78.1,17.1 | 78.1,17.1 R24.2 R87.2 | C50.1 74.95,18.25 76.1,17.1 78.1,17.1 | 74.95,39 78.2,39 R23.2 R22.2 R78.2 R84.2
  Top 0.5: 25,60.65 C37.1 25.05,61.45 24.85,61.65 21.6,61.65 21.45,61.65 20.75,62.35 20.75,64.25
  Top 1: 20.75,64.25 23.5,67 23.5,69.9 27.2,73.6 v28.6,73.6 v29.4,73.6 v30.2,73.6 v31,73.6 v31.8,73.6 | v67.9,73.6 v68.7,73.6 v69.5,73.6 v70.3,73.6 v71.1,73.6 72.5,73.6 75.9,70.2 75.9,66.4 77.1,65.2 77.1,64 77.1,62.4 75.3,60.6 75.3,60 | C64.+ X1.4
  Bottom 1: 56.3,73.6 v31.8,73.6 v28.6,73.6 | 56.3,73.6 v67.9,73.6 v71.1,73.6 | 56.3,73.6 X1.4

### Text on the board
Top: Hit | OR | C | T | T | C | T1 | T3 | T4 | T2 | V | V | HV | Liverpool University I.T. May 2013 | Quad Pixel Rigid Board V2.2
tValues: + | +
